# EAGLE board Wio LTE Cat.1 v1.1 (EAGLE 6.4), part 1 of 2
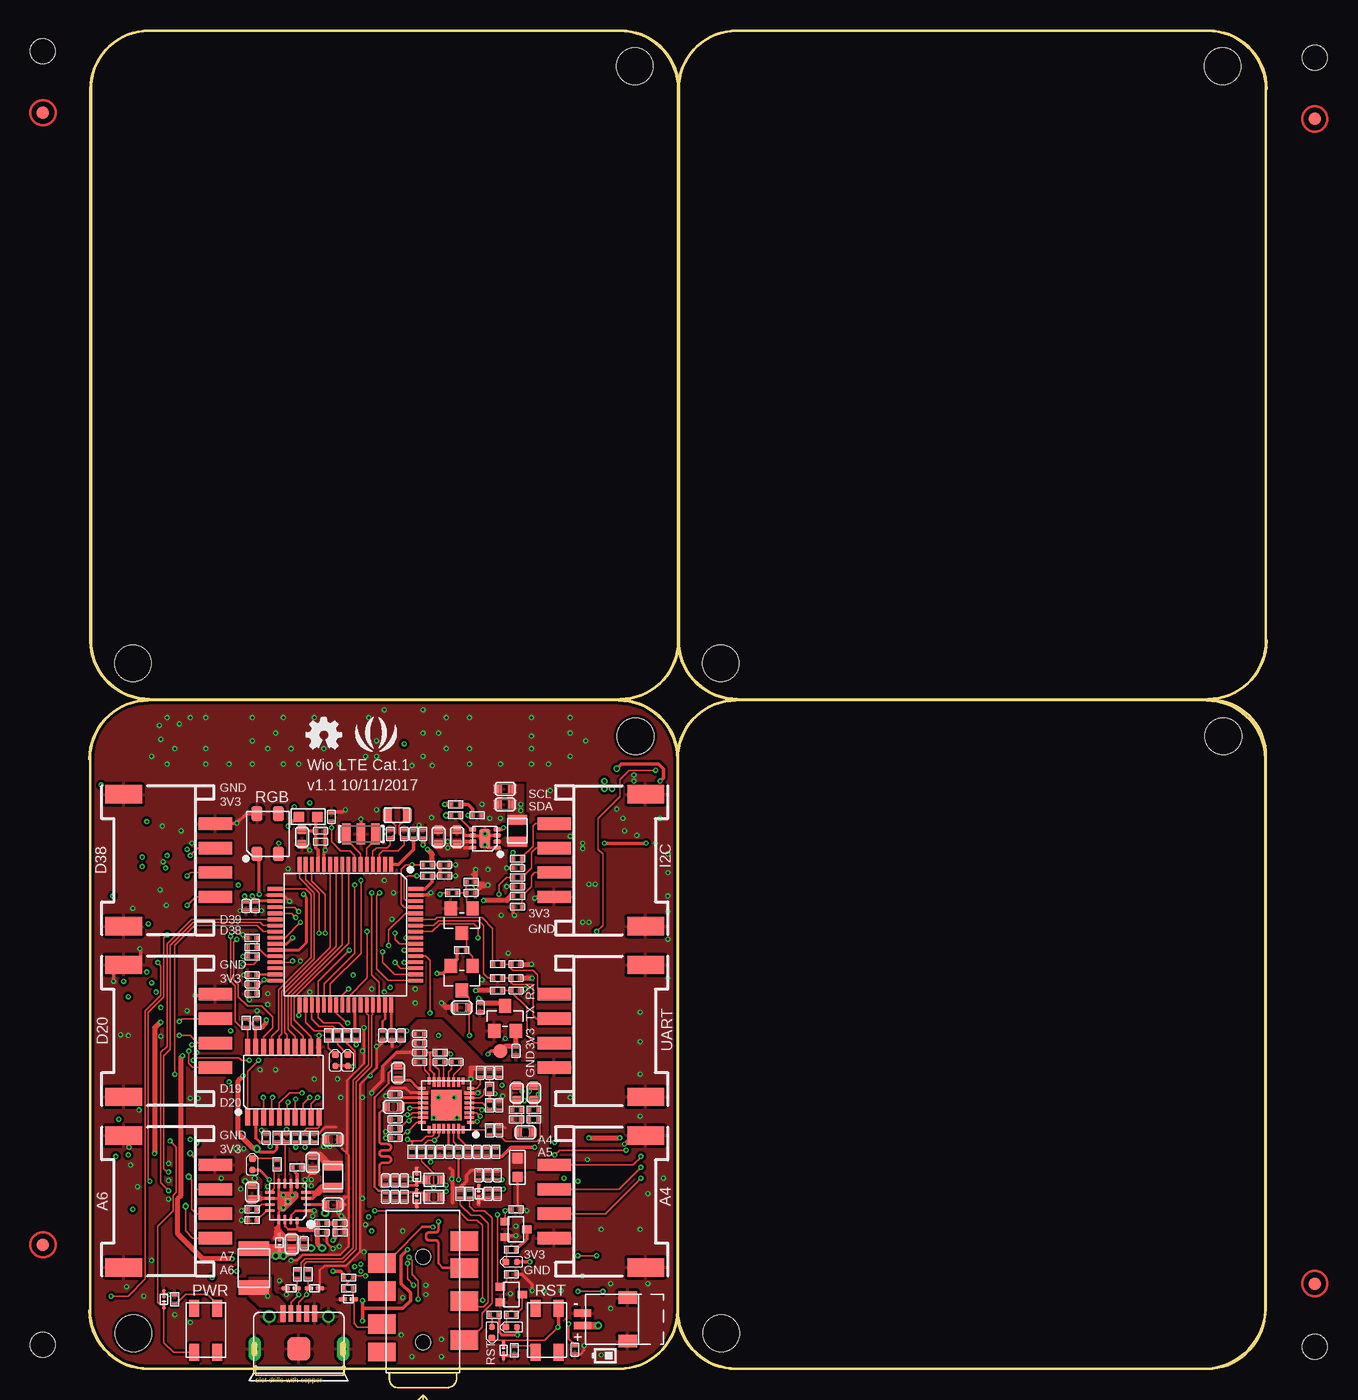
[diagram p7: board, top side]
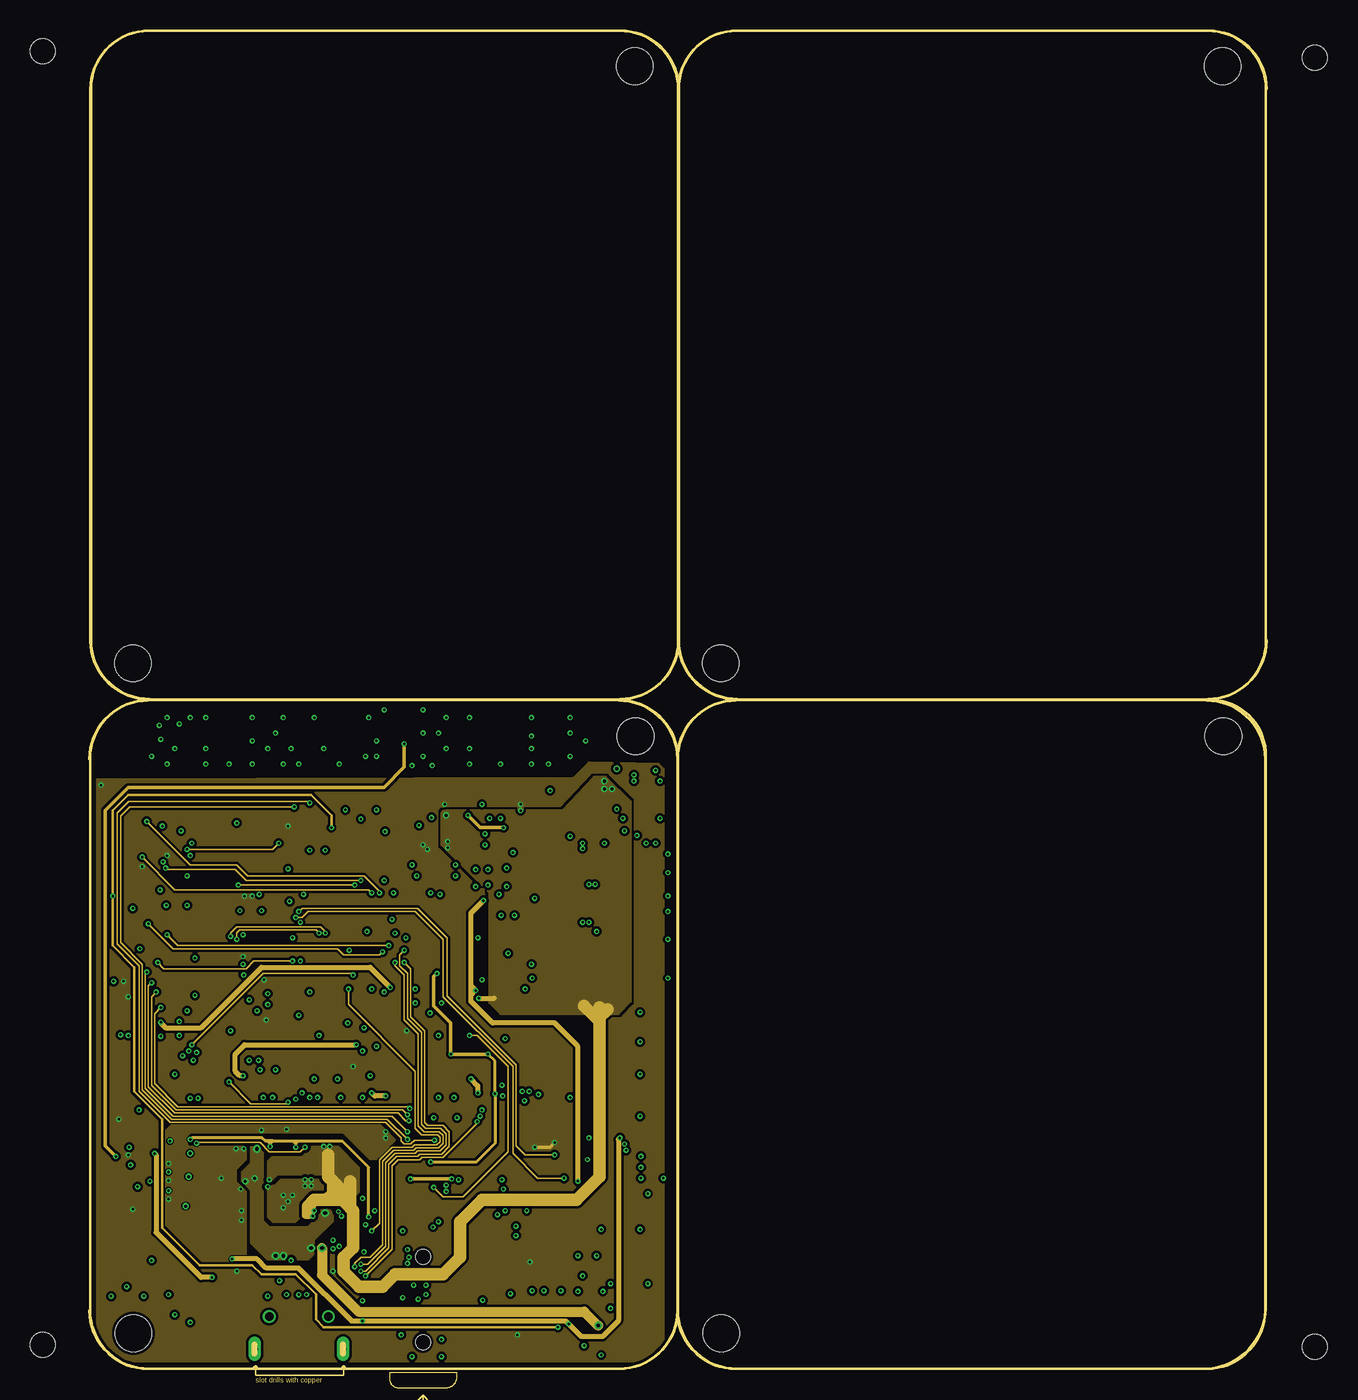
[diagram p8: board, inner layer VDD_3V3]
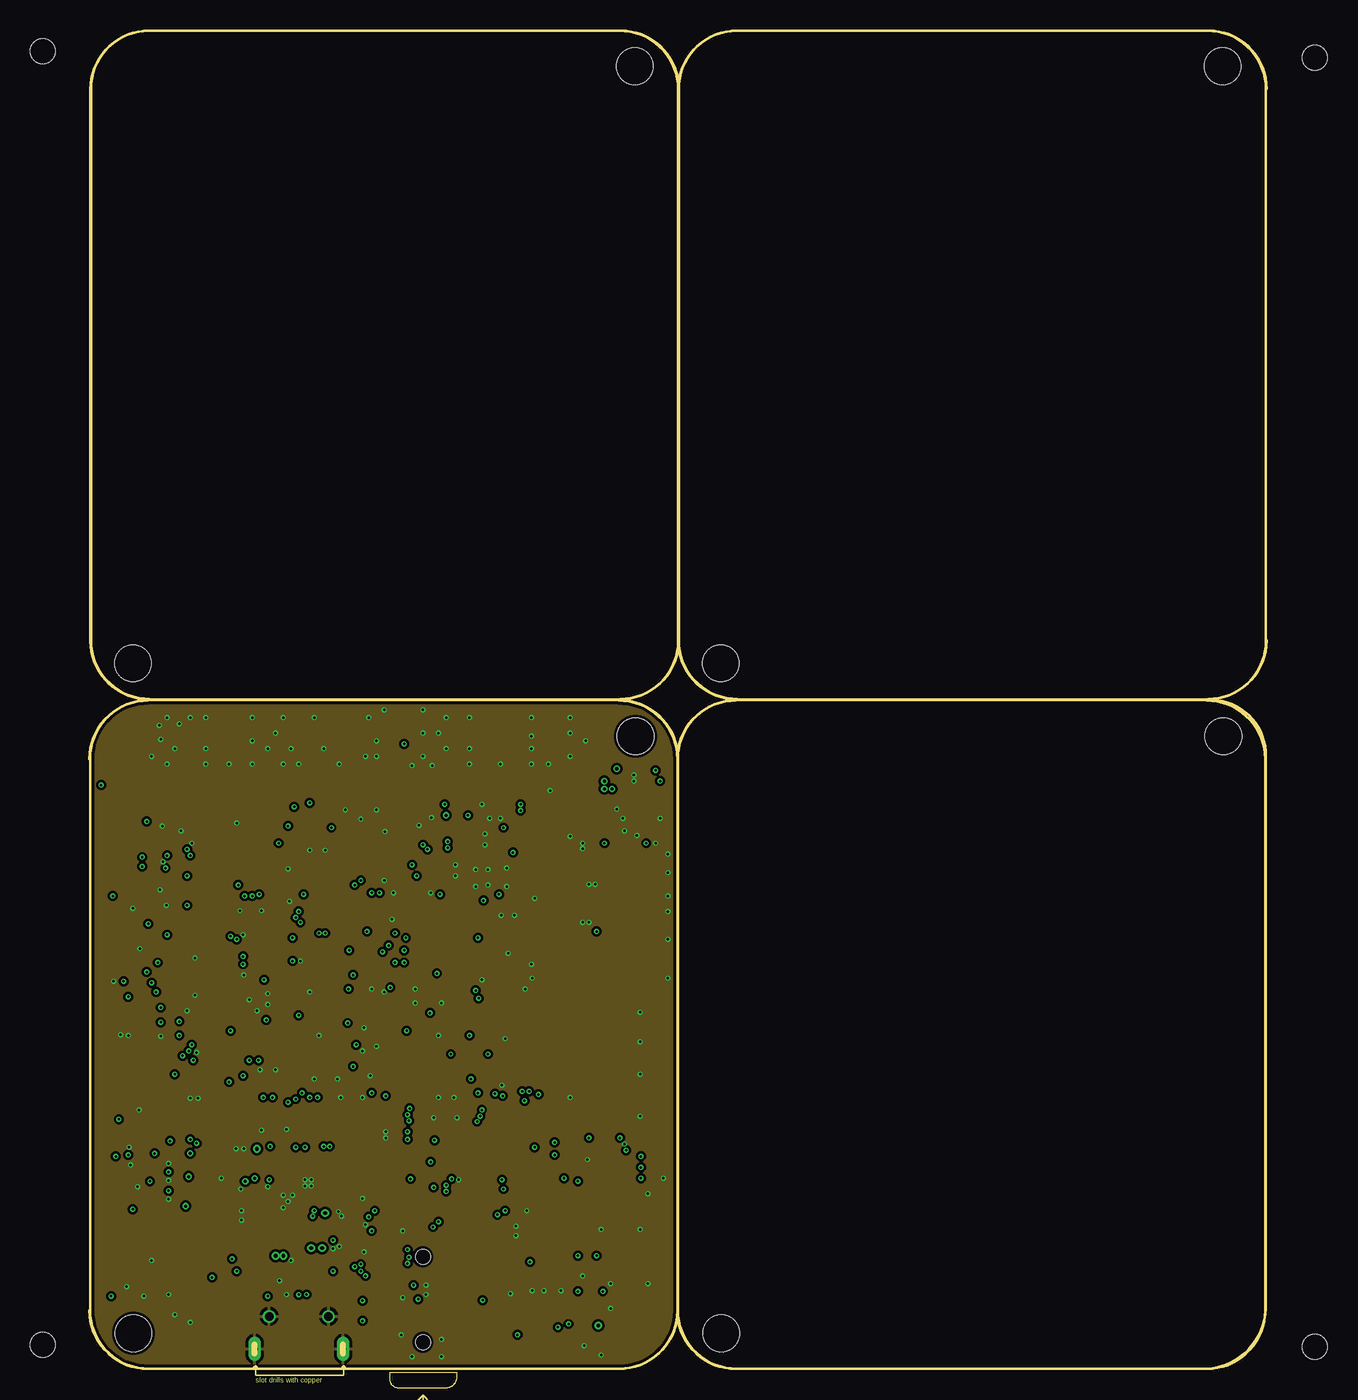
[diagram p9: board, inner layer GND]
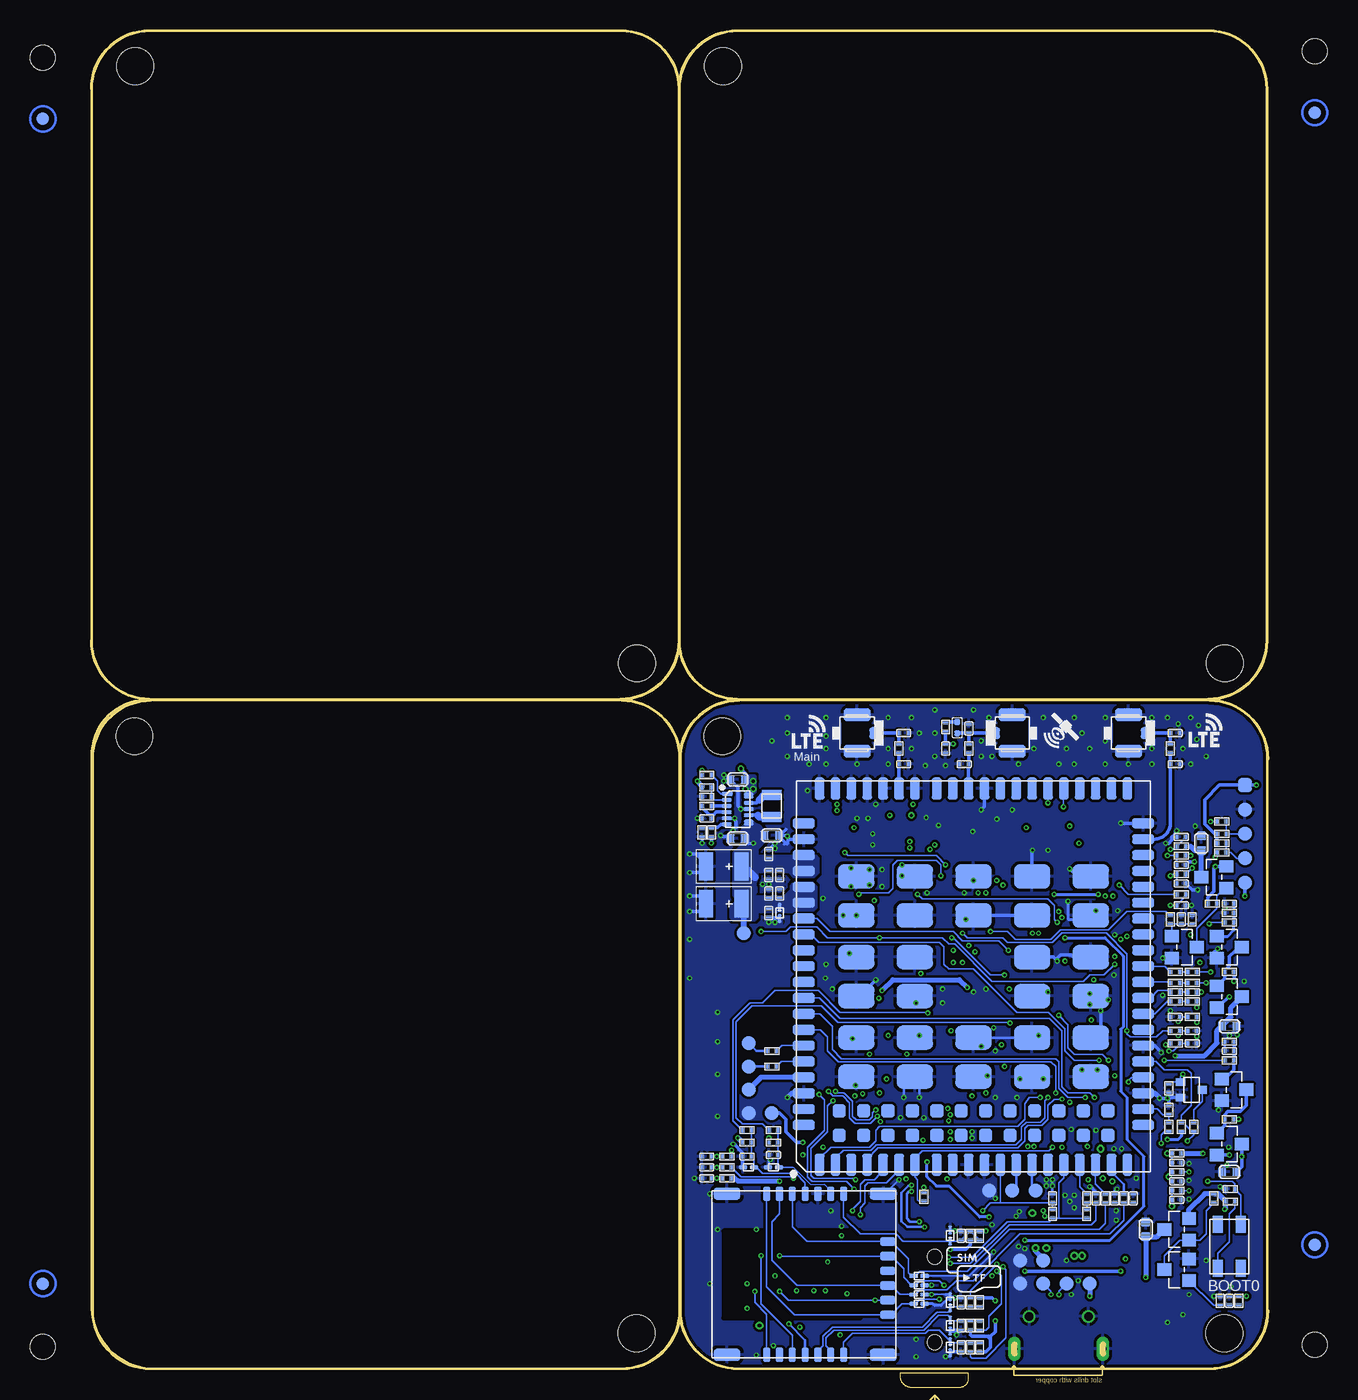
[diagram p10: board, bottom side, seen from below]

Size 96.39 x 109.6 mm. Coordinates in mm from the lower left corner, seen from the top.
Outline: 71 segments
Copper layers (1*2*15*16): Top 0.035mm / dielectric 0.2mm / VDD_3V3 0.0175mm / dielectric 0.3mm / GND 0.0175mm / dielectric 0.2mm / Bottom 0.035mm
Design rules "SeeedStudio_4layer_DRU_no_angle_20140221 *": minimum track width 1mil, minimum drill 8mil, track to track 4mil, track to pad 4mil, pad to pad 4mil, via to via 4mil, smd to smd 0mil, copper to edge 10mil, drill to drill 8mil, minimum pad ring 3mil, minimum via ring 3mil, stop-mask expansion 4mil, vias tented up to drill 25mil, thermal gap 10mil
Holes 3 mm at 3.6,2.92 44.7,51.82 51.74,2.92 92.84,51.82 92.79,106.68 51.69,57.78 44.66,106.68 3.56,57.78
Holes 2.03 mm at -3.81,1.98 -3.81,107.9 100.33,107.36 100.33,1.83
tRestrict: area 31.1,31.4 to 31.9,32.8; area 19.2,15.4 to 20.7,16.1; area 34.3,43.8 to 35.8,44.3
bRestrict: area 39.9,45.7 to 41.3,46.5; area 32.1,47.4 to 32.4,47.8; area 33.3,47.4 to 33.7,47.8; area 34.5,47.4 to 35.1,47.6; area 35.9,47.4 to 36.2,47.6; area 23.7,16.5 to 24,16.9

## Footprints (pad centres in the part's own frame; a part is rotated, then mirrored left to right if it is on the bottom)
U-FL3P-SMD-2.6X2.6X1.0MM = smd 1.05 x 1: D -1.524,0 | smd 2.2 x 1.05: GND1 0,1.5; GND2 0,-1.5
C0402 = smd 0.508 x 0.385: 1 0,0.383; 2 0,-0.383
C0603 = smd 0.762 x 0.696: 1 0,0.602; 2 0,-0.602
AVX-B = smd 1.143 x 2.286: + -1.46,0; - 1.46,0
SOD-923 = smd 0.7 x 0.3: 1 -0.45,0; 2 0.45,0
LED-0402 = smd 0.5 x 0.5: + -0.463,0 | smd 0.58 x 0.58: - 0.468,0
F1210 = smd 1.2 x 2.5: 1 -1.6,0; 2 1.6,0
HW2-SMD-1.0-90D = smd 1.524 x 1.016: 3 -3.429,1.778; 4 -3.429,-1.778 | smd 1.397 x 0.635: + 0.254,0.508; - 0.254,-0.508
SIM+TF-24P-SMD-1.2-15.05X13.66X2.5MM = smd 1.2 x 0.6: P1 0,3.26; P2 0,4.31; P3 0,5.36; P5 13.2,3.26; P6 13.2,4.31; P7 13.2,5.36; T1 13.2,9.56; T2 13.2,8.51; T3 13.2,7.46; T4 13.2,6.41; T5 0,6.41; T6 0,7.46; T7 0,8.51; T8 0,9.56 | smd 0.7 x 1.2: P1B 9.91,13.17; P2B 7.51,13.17; P3B 3.91,13.17; P5B 8.71,13.17; P6B 6.31,13.17; P7B 5.11,13.17 | smd 1 x 2.2: PAD 0,0; PAD1 0,12.8; PAD2 13.2,0; PAD3 13.2,12.8
AUDIO8P-SMD-3.5-14.5X6.1X4.0MM = smd 1.6 x 2.25: 1 3.9,-3.375; 2 7.1,-3.375; 3 9.8,-3.375; 4 10.2,3.375; 6 5.2,3.375; 7 7.9,3.375; 8 12,-3.375 | smd 1.5 x 2.25: 5 2.9,3.375 | hole 1.2: 3.7,0; 10.7,0
H5-SMD-2.0-TEST = smd 1.143 x 1.143: 1 0,4; 2 0,2; 3 0,0; 4 0,-2; 5 0,-4
MICRO-USB5+5P-SMD-0.65-7.2X5.06MM = smd 0.4 x 1.35: 1 -1.3,2.875; 2 -0.65,2.875; 3 0,2.875; 4 0.65,2.875; 5 1.3,2.875 | smd 1.9 x 1.9: P1 0,0 | drill 0.508 pad 1.016 long: P3 -3.625,0; P4 3.625,0 | drill 0.7: P5 -2.425,2.65; P6 2.425,2.65
HW4-SMD-2.0-90D = smd 1.01 x 2.74: 1 -3,-0.1; 2 -1,-0.1; 3 1,-0.1; 4 3,-0.1 | smd 1.5 x 3: SS1 -5.4,7.4; SS2 5.4,7.4
SW4P-SMD-4.5X3.2X2.5MM = smd 1.4 x 0.8: 1 -1.8,-0.94; 2 1.8,-0.94; 3 1.8,0.94; 4 -1.8,0.94
L0402 = smd 0.5 x 0.5: 1 -0.463,0; 2 0.463,0
L201610 = smd 0.8 x 1.6: 1 -0.9,0; 2 0.9,0
L0603 = smd 0.889 x 0.889: 1 -0.762,0; 2 0.762,0
LED4-1.75-3.7X3.5X0.95MM = smd 1.2 x 0.9: 1 -1.65,0.875; 2 -1.65,-0.875; 3 1.65,-0.875; 4 1.65,0.875
ROUND-MARK-1.0 = smd 1.016 x 1.016: P$1 0,0
SOT-323 = smd 0.635 x 0.762: 1 -0.635,-0.889; 2 0.635,-0.889; 3 0,0.889
SOT-23 = smd 1.016 x 1.143: 1 -0.889,-1.016; 2 0.889,-1.016; 3 0,1.016
R0402 = smd 0.508 x 0.385: 1 0,0.383; 2 0,-0.383
R0603 = smd 0.762 x 0.696: 1 0,0.602; 2 0,-0.602
R0603' = smd 0.889 x 0.889: 1 0,0.762; 2 0,-0.762
TP-D45MIL = smd 1.143 x 1.143: T 0,0
MODULE144P-1.3-32X29X2.4MM = smd 1.8 x 0.8: 1 -15.4,12.6; 2 -15.4,11.3; 3 -15.4,10; 4 -15.4,8.7; 5 -15.4,7.4; 6 -15.4,6.1; 7 -15.4,4.8; 8 -15.4,0.4; 9 -15.4,-0.9; 10 -15.4,-2.2; 11 -15.4,-3.5; 12 -15.4,-4.8; 13 -15.4,-6.1; 14 -15.4,-7.4; 15 -15.4,-8.7; 16 -15.4,-10; 17 -15.4,-11.3; 18 -15.4,-12.6; 37 15.4,-12.6; 38 15.4,-11.3; 39 15.4,-10; 40 15.4,-8.7; 41 15.4,-7.4; 42 15.4,-6.1; 43 15.4,-4.8; 44 15.4,-3.5; 45 15.4,-2.2; 46 15.4,-0.9; 47 15.4,0.4; 48 15.4,4.8; 49 15.4,6.1; 50 15.4,7.4; 51 15.4,8.7; 52 15.4,10; 53 15.4,11.3; 54 15.4,12.6; 141 -15.4,3; 142 -15.4,1.7; 143 15.4,1.7; 144 15.4,3 | smd 0.8 x 1.8: 19 -9.55,-13.9; 20 -8.25,-13.9; 21 -6.95,-13.9; 22 -5.65,-13.9; 23 -4.35,-13.9; 24 -3.05,-13.9; 25 -1.75,-13.9; 26 -0.45,-13.9; 27 0.85,-13.9; 28 2.15,-13.9; 29 3.45,-13.9; 30 4.75,-13.9; 31 6.05,-13.9; 32 7.35,-13.9; 33 8.65,-13.9; 34 9.95,-13.9; 35 11.25,-13.9; 36 12.55,-13.9; 55 12.55,13.9; 56 11.25,13.9; 57 9.95,13.9; 58 8.65,13.9; 59 7.35,13.9; 60 6.05,13.9; 61 4.75,13.9; 62 3.45,13.9; 63 2.15,13.9; 64 0.85,13.9; 65 -0.45,13.9; 66 -1.75,13.9; 67 -3.05,13.9; 68 -4.35,13.9; 69 -5.65,13.9; 70 -6.95,13.9; 71 -8.25,13.9; 72 -9.55,13.9; 113 -10.85,13.9; 114 -12.15,13.9; 115 -10.85,-13.9; 116 -12.15,-13.9 | smd 2 x 3: 85 8.2,9.6; 86 8.2,4.8; 87 8.2,0; 88 8.2,-4.8; 89 8.2,-9.6; 90 5,9.6; 91 5,4.8; 92 5,0; 93 5,-4.8; 94 5,-9.6; 95 1.6,9.6; 96 1.6,4.8; 97 1.6,-4.8; 98 1.6,-9.6; 99 -1.6,9.6; 100 -1.6,4.8; 101 -1.6,-4.8; 102 -1.6,-9.6; 103 -5,9.6; 104 -5,4.8; 105 -5,0; 106 -5,-4.8; 107 -5,-9.6; 108 -8.2,9.6; 109 -8.2,4.8; 110 -8.2,0; 111 -8.2,-4.8; 112 -8.2,-9.6 | smd 1.1 x 1.1: 117 -11,11; 118 -11,9; 119 -11,7; 120 -11,5; 121 -11,3; 122 -11,1; 123 -11,-1; 124 -11,-3; 125 -11,-5; 126 -11,-7; 127 -11,-9; 128 -11,-11; 129 -13,11; 130 -13,9; 131 -13,7; 132 -13,5; 133 -13,3; 134 -13,1; 135 -13,-1; 136 -13,-3; 137 -13,-5; 138 -13,-7; 139 -13,-9; 140 -13,-11
LQFP64 = smd 0.3 x 1.2: 1 -3.75,-5.75; 2 -3.25,-5.75; 3 -2.75,-5.75; 4 -2.25,-5.75; 5 -1.75,-5.75; 6 -1.25,-5.75; 7 -0.75,-5.75; 8 -0.25,-5.75; 9 0.25,-5.75; 10 0.75,-5.75; 11 1.25,-5.75; 12 1.75,-5.75; 13 2.25,-5.75; 14 2.75,-5.75; 15 3.25,-5.75; 16 3.75,-5.75; 33 3.75,5.75; 34 3.25,5.75; 35 2.75,5.75; 36 2.25,5.75; 37 1.75,5.75; 38 1.25,5.75; 39 0.75,5.75; 40 0.25,5.75; 41 -0.25,5.75; 42 -0.75,5.75; 43 -1.25,5.75; 44 -1.75,5.75; 45 -2.25,5.75; 46 -2.75,5.75; 47 -3.25,5.75; 48 -3.75,5.75 | smd 1.2 x 0.3: 17 5.75,-3.75; 18 5.75,-3.25; 19 5.75,-2.75; 20 5.75,-2.25; 21 5.75,-1.75; 22 5.75,-1.25; 23 5.75,-0.75; 24 5.75,-0.25; 25 5.75,0.25; 26 5.75,0.75; 27 5.75,1.25; 28 5.75,1.75; 29 5.75,2.25; 30 5.75,2.75; 31 5.75,3.25; 32 5.75,3.75; 49 -5.75,3.75; 50 -5.75,3.25; 51 -5.75,2.75; 52 -5.75,2.25; 53 -5.75,1.75; 54 -5.75,1.25; 55 -5.75,0.75; 56 -5.75,0.25; 57 -5.75,-0.25; 58 -5.75,-0.75; 59 -5.75,-1.25; 60 -5.75,-1.75; 61 -5.75,-2.25; 62 -5.75,-2.75; 63 -5.75,-3.25; 64 -5.75,-3.75
QFN32G-0.4-4X4MM = smd 0.6 x 0.25: 1 -2,1.4; 8 -2,-1.4; 17 2,-1.4; 24 2,1.4 | smd 0.8 x 0.25: 2 -1.9,1; 3 -1.9,0.6; 4 -1.9,0.2; 5 -1.9,-0.2; 6 -1.9,-0.6; 7 -1.9,-1; 18 1.9,-1; 19 1.9,-0.6; 20 1.9,-0.2; 21 1.9,0.2; 22 1.9,0.6; 23 1.9,1 | smd 0.25 x 0.6: 9 -1.4,-2; 16 1.4,-2; 25 1.4,2; 32 -1.4,2 | smd 0.25 x 0.8: 10 -1,-1.9; 11 -0.6,-1.9; 12 -0.2,-1.9; 13 0.2,-1.9; 14 0.6,-1.9; 15 1,-1.9; 26 1,1.9; 27 0.6,1.9; 28 0.2,1.9; 29 -0.2,1.9; 30 -0.6,1.9; 31 -1,1.9 | smd 2.5 x 2.5: PAD 0,0
QFN16G-0.5-3X3MM@1 = smd 0.65 x 0.28: 1 -1.575,0.75; 2 -1.575,0.25 | smd 0.85 x 0.28: 3 -1.475,-0.25; 4 -1.475,-0.75; 9 1.475,-0.75; 10 1.475,-0.25; 11 1.475,0.25; 12 1.475,0.75 | smd 0.28 x 0.85: 5 -0.75,-1.475; 6 -0.25,-1.475; 7 0.25,-1.475; 8 0.75,-1.475; 13 0.75,1.475; 14 0.25,1.475 | smd 0.28 x 0.65: 15 -0.25,1.575; 16 -0.75,1.575 | smd 0.508 x 0.508: PAD 0,0
DFN8G-0.5-2X2MM = smd 0.6 x 0.3: 1 -1,0.75; 2 -1,0.25; 3 -1,-0.25; 4 -1,-0.75; 5 1,-0.75; 6 1,-0.25; 7 1,0.25; 8 1,0.75 | smd 0.9 x 1.6: 9 0,0
QFN11-0.5-2X3MM = smd 0.9 x 0.3: 1 -0.85,1.25 | smd 0.8 x 0.3: 2 -0.9,0.75; 3 -0.9,0.25; 4 -0.9,-0.25; 5 -0.9,-0.75; 6 -0.9,-1.25; 8 0.9,-0.5; 9 0.9,0; 10 0.9,0.5 | smd 0.8 x 0.5: 7 0.9,-1.1; 11 0.9,1.1
TSSOP20-0.65-6.5X4.4MM = smd 0.4 x 1.35: 1 -2.925,-2.875; 2 -2.275,-2.875; 3 -1.625,-2.875; 4 -0.975,-2.875; 5 -0.325,-2.875; 6 0.325,-2.875; 7 0.975,-2.875; 8 1.625,-2.875; 9 2.275,-2.875; 10 2.925,-2.875; 11 2.91,2.875; 12 2.26,2.875; 13 1.61,2.875; 14 0.96,2.875; 15 0.325,2.875; 16 -0.325,2.875; 17 -0.975,2.875; 18 -1.625,2.875; 19 -2.275,2.875; 20 -2.925,2.875
X2-SMD-L2.0X1.2X0.55MM = smd 0.762 x 1.143: 1 -0.813,0; 2 0.813,0
RESONATOR3-SMD-3.6X1.3X0.8MM = smd 0.7 x 1.7: 1 -1.2,0; 2 0,0; 3 1.2,0

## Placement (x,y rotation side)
ANT1  [U-FL3P-SMD-2.6X2.6X1.0MM]  11.43,52.07 180 bottom
ANT2  [U-FL3P-SMD-2.6X2.6X1.0MM]  20.95,52.07 0 bottom
ANT4  [U-FL3P-SMD-2.6X2.6X1.0MM]  33.66,52.07 180 bottom
C1  4.7uF  [C0402]  13.34,32.26 90 top
C2  10uF  [C0402]  32,29.59 180 top
C3  10uF  [C0603]  19.94,13.46 90 top
C4  10uF  [C0603]  13.34,14.48 0 top
C5  100nF  [C0402]  40.01,38.93 0 bottom
C6  33pF  [C0402]  25.15,10.92 180 bottom
C7  100nF  [C0402]  17.59,10.29 0 top
C8  10uF  [C0603]  16.57,10.22 0 top
C9  DNP  [C0402]  29.84,49.53 270 bottom
C10  22pF  [C0402]  25.78,43.81 180 top
C11  22pF  [C0402]  24.64,43.81 180 top
C12  33pF  [C0402]  25.15,1.78 0 bottom
C13  22uF  [C0603]  43.43,48.26 90 bottom
C14  10pF  [C0402]  40.89,37.34 180 bottom
C15  22uF  [C0603]  40.64,43.69 90 bottom
C16  100nF  [C0402]  39.75,1.59 180 top
C17  33pF  [C0402]  25.15,5.46 180 bottom
C18  33pF  [C0402]  42.67,17.4 270 bottom
C19  33pF  [C0402]  14.1,13.97 180 bottom
C20  33pF  [C0402]  12.57,13.97 180 bottom
C21  33pF  [C0402]  11.05,13.97 180 bottom
C22  1uF  [C0402]  7.11,43.56 90 bottom
C23  100nF  [C0402]  19.81,45.21 180 top
C24  22uF  [C0603]  18.29,16.89 0 top
C25  1uF  [C0402]  19.05,11.18 90 top
C26  2.2uF  [C0402]  30.04,25.15 90 top
C27  2.2uF  [C0402]  28.7,25.15 90 top
C28  1uF  [C0603]  24.89,21.46 270 top
C29  1uF  [C0603]  25.27,24.26 180 top
C30  100nF  [C0402]  13.59,37.91 180 top
C31  1uF  [C0402]  12.83,37.91 180 top
C32  100nF  [C0402]  13.34,31.5 90 top
C33  2.2uF  [C0402]  25.02,22.48 270 top
C34  DNP  [C0402]  29.84,52.07 270 bottom
C35  4.7uF  [C0402]  27.05,27.43 90 top
C36  2.2uF  [C0402]  27.05,25.15 270 top
C37  4.7uF  [C0402]  33.53,19.56 0 top
C38  1uF  [C0402]  27.3,43.81 0 top
C39  100nF  [C0402]  26.54,43.81 0 top
C40  DNP  [C0402]  25.02,18.92 270 top
C41  DNP  [C0402]  25.02,19.68 270 top
C42  4.7uF  [C0402]  32,24.26 0 top
C43  100nF  [C0402]  27.05,26.67 90 top
C44  DNP  [C0402]  25.02,20.45 270 top
C45  33pF  [C0402]  27.05,25.91 90 top
C46  2.2uF  [C0402]  30.23,17.78 0 top
C47  2.2uF  [C0402]  28.7,17.78 180 top
C48  100nF  [C0402]  29.46,17.78 0 top
C49  4.7uF  [C0402]  32.51,17.78 180 top
C50  100nF  [C0402]  31.75,17.78 180 top
C51  33pF  [C0402]  30.99,17.78 180 top
C52  4.7uF  [C0402]  33.53,24.26 0 top
C53  100nF  [C0402]  32.77,24.26 0 top
C54  4.7uF  [C0402]  33.53,21.59 0 top
C55  22uF  [C0603]  43.43,43.43 270 bottom
C56  1uF  [C0402]  45.97,45.09 90 bottom
C57  33pF  [C0402]  7.11,39.75 90 bottom
C58  100nF  [C0402]  17.65,12.7 180 bottom
C59  33pF  [C0402]  17.65,13.97 180 bottom
C60  33pF  [C0402]  40.51,17.53 270 bottom
C61  33pF  [C0402]  25.15,3.56 0 bottom
C62  33pF  [C0402]  7.11,37.97 90 bottom
C63  33pF  [C0402]  7.11,41.27 90 bottom
C64  33pF  [C0402]  6.22,27.69 90 bottom
C65  100nF  [C0402]  14.48,18.92 0 top
C66  100nF  [C0402]  29.08,40.39 270 top
C67  100nF  [C0402]  7.11,36.83 180 bottom
C68  1uF  [C0402]  13.34,30.73 90 top
C70  100nF  [C0402]  24.77,27.3 180 top
C71  1uF  [C0402]  25.53,27.3 180 top
C74  33pF  [C0402]  40.89,38.93 0 bottom
C75  100nF  [C0402]  29.08,41.27 270 top
C76  1uF  [C0402]  13.72,28.32 0 top
C77  220uF  [AVX-B]  44.58,38.1 180 bottom
C78  100nF  [C0402]  20.51,11.94 90 top
C79  10uF  [C0603]  3.17,28.07 90 bottom
C80  10uF  [C0603]  35.69,19.37 90 top
C81  2.2uF  [C0603]  36.39,22.61 180 top
C82  2.2uF  [C0603]  34.99,22.61 180 top
C83  4.7uF  [C0402]  33.4,15.88 0 top
C84  10pF  [C0402]  31.88,15.88 0 top
C85  33pF  [C0402]  32.64,15.88 0 top
C86  33pF  [C0402]  24.26,14.1 180 top
C87  10pF  [C0402]  25.02,15.43 180 top
C88  33pF  [C0402]  24.26,15.43 0 top
C89  10pF  [C0402]  25.02,14.1 180 top
C90  33pF  [C0402]  33.4,14.35 180 top
C91  100nF  [C0402]  3.17,38.1 270 bottom
C92  10uF  [C0603]  3.17,16.13 270 bottom
C93  100nF  [C0402]  3.17,26.04 270 bottom
C94  10pF  [C0402]  32.64,14.35 180 top
C95  DNP  [C0402]  7.62,49.53 270 bottom
C96  DNP  [C0402]  25.78,15.43 180 top
C97  DNP  [C0402]  25.78,14.1 180 top
C98  DNP  [C0402]  7.62,52.07 270 bottom
C99  DNP  [C0402]  24.89,49.53 90 bottom
C100  DNP  [C0402]  24.51,52.45 0 bottom
C101  DNP  [C0402]  26.42,50.8 180 bottom
C102  10uF  [C0603]  34.04,46.23 90 top
C103  10uF  [C0603]  28.57,43.56 0 top
C104  10uF  [C0603]  34.04,47.5 90 top
C105  10uF  [C0603]  30.1,43.56 0 top
C106  100nF  [C0402]  40.89,42.16 0 bottom
C107  10pF  [C0402]  40.89,40.45 180 bottom
C112  33pF  [C0402]  40.01,40.45 180 bottom
C113  220uF  [AVX-B]  44.58,41.15 180 bottom
C114  33pF  [C0402]  7.62,28.83 270 bottom
C115  33pF  [C0402]  6.22,26.67 90 bottom
C116  33pF  [C0402]  7.49,15.37 90 bottom
C117  33pF  [C0402]  7.49,16.89 90 bottom
C118  1uF  [C0402]  18.92,43.18 270 top
C119  100nF  [C0402]  18.92,44.07 270 top
C120  10uF  [C0402]  34.92,26.04 180 top
C125  4.7uF  [C0402]  24,27.3 180 top
C126  33pF  [C0402]  7.49,13.84 90 bottom
C127  33pF  [C0402]  34.92,32 90 top
C128  33pF  [C0402]  34.92,30.99 90 top
C129  33pF  [C0402]  34.92,33.15 90 top
C130  33pF  [C0402]  45.97,16.51 270 bottom
C131  33pF  [C0402]  45.97,15.62 270 bottom
C132  33pF  [C0402]  45.97,17.4 270 bottom
C133  33pF  [C0402]  35.05,39.5 270 top
C134  33pF  [C0402]  35.05,37.85 270 top
C135  33pF  [C0402]  35.05,41.02 270 top
C136  10uF  [C0603]  10.03,11.43 180 bottom
C137  100nF  [C0402]  3.17,5.59 180 bottom
C138  22uF  [C0603]  19.94,18.8 90 top
C139  22uF  [C0603]  17.4,43.56 0 top
C140  10uF  [C0603]  5.46,43.05 180 bottom
C142  10uF  [C0603]  30.48,29.59 270 top
C143  100nF  [C0402]  31.24,38.99 90 top
D1  DF2S6.8FS  [SOD-923]  15.56,10.35 90 top
D3  DF2S6.8FS  [SOD-923]  16.51,6.6 180 top
D5  DF2S6.8FS  [SOD-923]  18.41,6.6 0 top
D6  GREEN  [LED-0402]  21.15,25.27 90 top
D7  ESD;DF2S6.8FS  [SOD-923]  26.04,1.78 270 bottom
D8  ESD;DF2S6.8FS  [SOD-923]  28.57,6.86 0 bottom
D9  ESD;DF2S6.8FS  [SOD-923]  26.8,15.75 90 top
D10  ESD;DF2S6.8FS  [SOD-923]  28.57,7.62 0 bottom
D11  ESD;DF2S6.8FS  [SOD-923]  28.57,6.1 0 bottom
D12  ESD;DF2S6.8FS  [SOD-923]  28.57,5.33 0 bottom
D13  ESD;DF2S6.8FS  [SOD-923]  26.8,13.97 270 top
D14  RED  [LED-0402]  32.96,2.98 270 top
D15  ESD;DF2S6.8FS  [SOD-923]  31.88,14.35 270 top
D16  GREEN  [LED-0402]  13.34,16.76 90 top
D17  GREEN  [LED-0402]  20.13,25.27 90 top
D18  ESD;DF2S6.8FS  [SOD-923]  21.21,5.71 180 top
D19  ESD;DF2S6.8FS  [SOD-923]  40.51,16.51 180 bottom
D20  ESD;DF2S6.8FS  [SOD-923]  42.55,16.51 180 bottom
D21  ESD;DF2S6.8FS  [SOD-923]  26.04,10.92 90 bottom
D22  ESD;DF2S6.8FS  [SOD-923]  26.04,5.46 90 bottom
D23  ESD;DF2S6.8FS  [SOD-923]  26.04,3.56 270 bottom
D24  RED  [LED-0402]  34.54,3.43 180 top
D25  RED  [LED-0402]  34.54,8.76 180 top
D26  ESD;DF2S6.8FS  [SOD-923]  6.1,5.71 90 top
D27  ESD;DF2S6.8FS  [SOD-923]  33.91,1.52 270 top
D28  DNP  [SOD-923]  40.01,37.34 270 bottom
F1  2A/6V  [F1210]  13.46,8.26 90 top
FR1  SEEEDSTUDIO-OPEN-SCH-FRAME  [SEEEDSTUDIO-PCB-FRAME]  not placed on the board
FR2  SEEEDSTUDIO-OPEN-SCH-FRAME  [SEEEDSTUDIO-PCB-FRAME]  not placed on the board
FR3  SEEEDSTUDIO-OPEN-SCH-FRAME  [SEEEDSTUDIO-PCB-FRAME]  not placed on the board
FR4  SEEEDSTUDIO-OPEN-SCH-FRAME  [SEEEDSTUDIO-PCB-FRAME]  not placed on the board
FR5  SEEEDSTUDIO-OPEN-SCH-FRAME  [SEEEDSTUDIO-PCB-FRAME]  not placed on the board
FR6  SEEEDSTUDIO-OPEN-SCH-FRAME  [SEEEDSTUDIO-PCB-FRAME]  not placed on the board
FR7  SEEEDSTUDIO-OPEN-SCH-FRAME  [SEEEDSTUDIO-PCB-FRAME]  not placed on the board
FR8  SEEEDSTUDIO-OPEN-SCH-FRAME  [SEEEDSTUDIO-PCB-FRAME]  not placed on the board
FR9  SEEEDSTUDIO-OPEN-SCH-FRAME  [SEEEDSTUDIO-PCB-FRAME]  not placed on the board
FR10  SEEEDSTUDIO-OPEN-SCH-FRAME  [SEEEDSTUDIO-PCB-FRAME]  not placed on the board
J1  JST-2P-SMD-90D  [HW2-SMD-1.0-90D]  40.64,4.06 180 top
J2  [SIM+TF-24P-SMD-1.2-15.05X13.66X2.5MM]  44.32,14.35 270 bottom
J3  [AUDIO8P-SMD-3.5-14.5X6.1X4.0MM]  27.3,-1.52 90 top
J4  [H5-SMD-2.0-TEST]  1.91,43.81 0 bottom
J10  USB  [MICRO-USB5+5P-SMD-0.65-7.2X5.06MM]  17.14,1.65 0 top
J11  D38  [HW4-SMD-2.0-90D]  10.21,41.66 90 top
J12  D20  [HW4-SMD-2.0-90D]  10.21,27.69 90 top
J13  A6  [HW4-SMD-2.0-90D]  10.21,13.72 90 top
J14  I2C  [HW4-SMD-2.0-90D]  38.15,41.66 270 top
J15  URAT  [HW4-SMD-2.0-90D]  38.15,27.69 270 top
J16  A4  [HW4-SMD-2.0-90D]  38.15,13.72 270 top
K1  KEY  [SW4P-SMD-4.5X3.2X2.5MM]  3.17,10.03 270 bottom
K3  KEY  [SW4P-SMD-4.5X3.2X2.5MM]  37.47,3.17 90 top
K4  KEY  [SW4P-SMD-4.5X3.2X2.5MM]  9.53,3.17 270 top
L1  47nH  [L0402]  25.46,52.51 90 bottom
L2  470nH  [L201610]  35.05,44.07 90 top
L3  1uH  [L201610]  40.64,46.1 270 bottom
L6  2.2uH  [L201610]  19.94,15.75 90 top
L12  30R/3000mA  [L0603]  17.91,45.21 0 top
LED2  RGB-SK6812MINI  [LED4-1.75-3.7X3.5X0.95MM]  14.61,43.81 270 top
P1  [ROUND-MARK-1.0]  not placed on the board
P2  [ROUND-MARK-1.0]  not placed on the board
P3  [ROUND-MARK-1.0]  not placed on the board
P4  [ROUND-MARK-1.0]  not placed on the board
P5  [ROUND-MARK-1.0]  not placed on the board
P6  [ROUND-MARK-1.0]  not placed on the board
P7  [ROUND-MARK-1.0]  not placed on the board
P8  [ROUND-MARK-1.0]  not placed on the board
Q1  2N7002KW  [SOT-323]  6.29,22.86 270 bottom
Q2  CJ3407A  [SOT-23]  7.49,11.43 90 bottom
Q3  2N7002  [SOT-23]  7.49,8.13 90 bottom
Q4  CJ3407A  [SOT-23]  4.45,40.26 90 bottom
Q5  2N7002  [SOT-23]  6.86,34.54 270 bottom
Q6  CJ3407A  [SOT-23]  30.48,32 180 top
Q7  2N7002  [SOT-23]  30.48,36.7 180 top
Q9  2N7002KW  [SOT-323]  34.54,6.1 270 top
Q10  2N7002KW  [SOT-323]  34.92,11.43 270 top
Q13  CJ3407A  [SOT-23]  3.17,30.48 270 bottom
Q14  2N7002  [SOT-23]  3.17,34.54 270 bottom
Q15  CJ3407A  [SOT-23]  3.17,18.41 270 bottom
Q16  2N7002  [SOT-23]  2.79,22.86 270 bottom
R1  0R  [R0402]  7.62,30.1 270 bottom
R2  0R  [R0402]  7.62,30.86 270 bottom
R3  0R  [R0402]  7.62,31.62 270 bottom
R4  0R  [R0402]  7.62,32.51 270 bottom
R5  0R  [R0402]  24.38,1.78 0 bottom
R6  0R  [R0402]  7.11,42.8 270 bottom
R8  1k  [R0402]  8,36.83 180 bottom
R9  22R  [R0402]  40.64,24.77 270 bottom
R10  22R  [R0402]  40.64,26.04 270 bottom
R11  4.7K  [R0402]  3.11,13.72 270 bottom
R12  100K  [R0402]  3.11,14.73 270 bottom
R13  0R  [R0402]  3.81,44.83 90 bottom
R14  0R  [R0402]  3.81,42.29 90 bottom
R15  DNP  [R0402]  3.81,43.81 270 bottom
R16  22R  [R0402]  17.02,7.75 180 top
R17  22R  [R0402]  17.91,7.75 180 top
R18  DNP  [R0402]  3.81,43.05 270 bottom
R19  2K  [R0402]  15.37,16.76 0 top
R20  2K  [R0402]  13.34,12.19 270 top
R21  2K  [R0402]  13.34,13.08 270 top
R22  0R  [R0402]  30.23,50.8 180 bottom
R23  15K  [R0402]  14.86,12.7 180 bottom
R24  0R  [R0402]  23.62,3.56 0 bottom
R25  22R  [R0402]  11.81,13.97 0 bottom
R26  22R  [R0402]  13.34,13.97 0 bottom
R27  22R  [R0402]  14.86,13.97 0 bottom
R28  1M  [R0402]  6.22,36.83 0 bottom
R29  0R  [R0402]  34.8,1.52 0 top
R30  0R  [R0402]  6.99,5.71 180 top
R31  4.7K  [R0402]  33.15,4.45 270 top
R32  0R  [R0402]  16.13,18.92 180 top
R33  DNP  [R0402]  15.37,18.92 180 top
R34  0R  [R0402]  17.02,16.51 90 top
R35  4.7K  [R0402]  27.69,40.39 90 top
R36  4.7K  [R0402]  27.69,41.27 90 top
R37  470R  [R0402]  6.1,19.81 0 bottom
R38  10K  [R0402]  8.13,22.99 180 bottom
R39  0R  [R0402]  6.22,32.51 90 bottom
R40  0R  [R0402]  6.22,31.62 90 bottom
R41  0R  [R0402]  6.22,30.86 90 bottom
R42  0R  [R0402]  6.22,30.1 90 bottom
R43  470R  [R0402]  20.32,27.3 0 top
R44  470R  [R0402]  19.56,27.3 0 top
R45  100K_1%  [R0402]  29.97,46.23 270 top
R46  10M  [R0402]  19.05,11.94 270 top
R47  10M  [R0402]  20.51,11.18 270 top
R48  0R  [R0402]  32.77,19.56 0 top
R49  22K_1%  [R0402]  31.75,45.34 270 top
R50  4.7K  [R0402]  26.42,17.78 0 top
R51  4.7K  [R0402]  27.18,17.78 0 top
R52  0R  [R0402]  28.7,25.91 90 top
R53  0R  [R0402]  27.94,17.78 0 top
R54  0R  [R0402]  32.77,22.92 0 top
R55  0R  [R0402]  32.77,21.59 180 top
R56  DNP  [R0402]  13.34,34.54 270 top
R57  0R  [R0402]  23.62,10.92 180 bottom
R58  0R  [R0402]  24.38,5.46 180 bottom
R60  0R  [R0402]  42.67,19.56 270 bottom
R61  0R  [R0402]  40.51,19.56 270 bottom
R62  DNP  [R0402]  24.38,3.56 180 bottom
R63  DNP  [R0402]  23.62,5.46 0 bottom
R64  DNP  [R0402]  42.67,18.54 90 bottom
R65  DNP  [R0402]  40.51,18.54 90 bottom
R70  1.5K  [R0402]  36.39,21.21 270 top
R71  1K  [R0402]  36.39,20.45 90 top
R72  1.5K  [R0402]  34.99,21.21 270 top
R73  1K  [R0402]  34.99,20.45 90 top
R74  10M  [R0402]  21.21,7.49 90 top
R75  0R  [R0402]  30.35,14.35 0 top
R76  DNP  [R0402]  23.62,1.78 180 bottom
R77  DNP  [R0402]  13.34,33.78 270 top
R78  1k  [R0402]  21.21,6.6 90 top
R79  DNP  [R0402]  45.97,47.62 90 bottom
R80  DNP  [R0402]  24.38,10.92 180 bottom
R81  4.7K  [R0402]  45.97,48.64 270 bottom
R82  0R  [R0402]  31.11,14.35 0 top
R83  0R  [R0603]  28.19,15.49 90 top
R84  0R  [R0603]  28.19,14.1 90 top
R85  DNP  [R0402]  7.11,19.81 0 bottom
R86  DNP  [R0402]  8.13,19.81 0 bottom
R87  DNP  [R0402]  8.13,21.21 0 bottom
R89  DNP  [R0402]  16.89,18.92 0 top
R90  0R  [R0402]  29.97,45.34 270 top
R91  470R  [R0402]  34.54,4.45 270 top
R92  DNP  [R0402]  34.54,7.75 270 top
R93  470R  [R0402]  34.54,9.78 270 top
R94  DNP  [R0402]  34.92,13.08 270 top
R95  0R  [R0402]  21.84,27.3 180 top
R96  10K  [R0402]  45.97,46.86 270 bottom
R97  200K1%  [R0402]  45.59,43.94 180 bottom
R98  30K1%  [R0402]  46.35,43.94 0 bottom
R99  100K  [R0402]  45.97,46.1 270 bottom
R100  10K  [R0402]  12.83,28.32 180 top
R101  10K  [R0402]  21.08,27.3 0 top
R102  1k  [R0402]  3.17,36.58 270 bottom
R103  470k  [R0402]  3.17,32.51 90 bottom
R104  1M  [R0402]  3.17,37.34 90 bottom
R105  1k  [R0402]  3.17,25.27 270 bottom
R106  470k  [R0402]  3.17,20.45 90 bottom
R107  1M  [R0402]  3.17,26.8 90 bottom
R108  0R  [R0603']  35.05,16.51 180 top
R109  0R  [R0402]  8,50.8 180 bottom
R110  0R  [R0402]  24.51,50.8 180 bottom
R111  0R  [R0402]  26.42,52.58 0 bottom
R112  DNP  [R0402]  13.34,35.31 90 top
R113  0R  [R0402]  7.11,42.04 90 bottom
R114  0R  [R0402]  7.11,40.51 90 bottom
R117  0R  [R0402]  7.11,38.86 270 bottom
R118  0R  [R0402]  6.22,28.83 90 bottom
R119  0R  [R0402]  7.62,27.69 270 bottom
R120  0R  [R0402]  7.62,26.67 270 bottom
R121  0R  [R0402]  7.49,17.65 90 bottom
R122  0R  [R0402]  7.49,16.13 90 bottom
R123  0R  [R0402]  7.49,14.61 90 bottom
R124  0R  [R0402]  44.32,15.62 90 bottom
R125  4.7K  [R0402]  17.65,18.92 0 top
R126  DNP  [R0402]  18.41,18.92 0 top
R127  0R  [R0402]  44.32,16.51 90 bottom
R128  0R  [R0402]  44.32,17.4 90 bottom
R129  0R  [R0402]  33.4,30.99 270 top
R130  0R  [R0402]  33.4,32 270 top
R131  0R  [R0402]  33.4,33.15 270 top
R132  0R  [R0402]  35.05,38.73 270 top
R133  0R  [R0402]  35.05,40.26 270 top
R134  0R  [R0402]  35.05,41.78 270 top
R135  1k  [R0402]  2.41,5.59 180 bottom
R136  470k  [R0402]  4.45,13.97 180 bottom
R137  1M  [R0402]  3.94,5.59 0 bottom
R139  470k  [R0402]  4.57,38.1 270 bottom
R141  DNP  [R0402]  28.19,14.1 180 bottom
R142  1k  [R0402]  29.72,38.99 270 top
R143  470k  [R0402]  30.48,34.29 270 top
R144  1M  [R0402]  31.24,39.88 270 top
R145  0R  [R0402]  33.27,17.78 0 top
TP1  [TP-D45MIL]  14.61,6.99 0 bottom
TP2  [TP-D45MIL]  20.32,6.99 0 bottom
TP3  [TP-D45MIL]  16.51,6.99 0 bottom
TP4  [TP-D45MIL]  18.41,6.99 0 bottom
TP5  [TP-D45MIL]  42.93,35.69 0 bottom
TP8  [TP-D45MIL]  33.66,26.04 180 top
TP12  [TP-D45MIL]  40.64,20.95 0 bottom
TP13  [TP-D45MIL]  42.55,22.86 180 bottom
TP14  [TP-D45MIL]  42.55,24.77 180 bottom
TP15  [TP-D45MIL]  42.55,26.67 180 bottom
TP16  [TP-D45MIL]  42.55,20.95 180 bottom
TP17  [TP-D45MIL]  20.95,14.61 180 bottom
TP18  [TP-D45MIL]  19.05,14.61 180 bottom
TP19  [TP-D45MIL]  22.86,14.61 180 bottom
TP20  [TP-D45MIL]  18.41,8.89 0 bottom
TP21  [TP-D45MIL]  20.32,8.89 0 bottom
U1  EC21-A  [MODULE144P-1.3-32X29X2.4MM]  24.13,32.13 90 bottom
U3  STM32F412RG  [LQFP64]  20.95,35.56 180 top
U4  ALC5616  [QFN32G-0.4-4X4MM]  29.21,21.59 180 top
U5  ETA6003  [QFN16G-0.5-3X3MM@1]  16.26,13.72 180 top
U6  ETA3410  [DFN8G-0.5-2X2MM]  32.38,43.43 180 top
U8  MP28164  [QFN11-0.5-2X3MM]  43.43,45.85 0 bottom
U9  TXS0108E  [TSSOP20-0.65-6.5X4.4MM]  15.88,23.5 0 top
U11  XC6206P182MR  [SOT-23]  34.04,28.7 0 top
U$97  [OSHW_FILLX100_NOTEXT]  17.78,50.8 0 top
U$98  [SEEED-SILK--TNAME-160*153MIL]  23.5,52.07 0 top
X1  32.768KHZ  [X2-SMD-L2.0X1.2X0.55MM]  25.21,45.34 180 top
X3  8M  [RESONATOR3-SMD-3.6X1.3X0.8MM]  22.23,43.81 180 top

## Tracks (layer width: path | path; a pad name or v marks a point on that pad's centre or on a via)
5V  (via drill 0.2 pad 0.41, 0.25 pad 0.51, 0.3 pad 0.64)
  Top 0.254: U5.2 C3.1 | v13.72,18.03 13.97,17.78 15.11,17.78 15.37,18.03 R33.1
  Top 0.305: R95.1 v21.84,26.54
  Top 0.406: v13.72,18.03 13.46,18.03 12.19,19.3 12.19,23.62 v12.57,24
  Top 0.508: F1.2 14.61,9.65 14.99,9.27 16,9.27 16.26,9.53 15.24,9.53 15.11,9.65
  Top 0.61: 16.6,9.9 14.22,9.9 F1.2 | D1.1 16.55,9.9 C8.2 16.6,9.9 | 16.6,9.9 C7.2 v18.16,9.91 | C3.1 19.34,12.73 v19.3,12.76
  VDD_3V3 0.406: v12.57,24 12.32,24 11.94,24.38 11.94,25.78 12.7,26.54 v21.84,26.54
  other vias: 15.24,9.27 15.88,9.27 13.53,15.62 12.76,15.37
  pour VDD_3V3 (isolate 0.254, no thermals): 18.92,13.08 19.68,13.08 19.94,12.83 19.94,12.06 18.41,10.54 18.41,9.4 17.91,8.89 14.61,8.89 13.21,10.29 13.21,14.61 12.83,14.99 12.45,15.37 12.45,16.13 13.21,16.89 13.21,18.29 13.34,18.41 13.97,18.41 14.22,18.16 14.22,12.19 14.73,11.68 17.91,11.68 18.8,12.57 18.8,12.95
  pour Top (isolate 0.254, no thermals): 13.72,14.73 12.95,14.73 12.45,15.24 12.45,15.62 12.7,15.88 13.72,15.88 14.1,15.49 14.1,14.86 13.97,14.73
A4  (via drill 0.2 pad 0.41)
  Top 0.127: U3.20 16.8,37.81 v17.14,37.47 | v43.94,17.91 38.48,17.91 v38.1,17.53
  VDD_3V3 0.127: v38.1,17.53 35.69,17.53 34.92,18.29 34.92,24.89 29.27,30.54 29.27,35.31 26.86,37.72 17.4,37.72 v17.14,37.47
  Bottom 0.127: R128.2 v43.94,17.91
A5  (via drill 0.2 pad 0.41)
  Top 0.127: U3.21 16.54,37.31 v16.89,36.96
  VDD_3V3 0.127: v16.89,36.96 17.4,36.96 17.91,37.47 26.68,37.47 28.96,35.19 28.96,30.48 34.67,24.77 34.67,17.65 36.7,15.62 v38.86,15.62
  Bottom 0.127: R127.2 43.18,15.75 38.99,15.75 v38.86,15.62
A6  (via drill 0.2 pad 0.41)
  Top 0.127: U3.22 8.36,36.81 6.35,34.8 6.35,26.42 5.84,25.91 5.84,15.24 v6.48,14.61
  Bottom 0.127: R123.2 v6.48,14.61
A7  (via drill 0.2 pad 0.41)
  Top 0.127: U3.23 14.24,36.31 13.97,36.58 8.51,36.58 6.6,34.67 6.6,26.16 6.1,25.65 6.1,16.38 6.35,16.13 v6.48,16.13
  Bottom 0.127: R122.2 v6.48,16.13
AGND  (via drill 0.2 pad 0.41)
  Top 0.203: C37.1 33.84,19.94 34.04,19.75
  Top 0.254: U4.7 31.8,22.59 v31.81,22.61 | U4.18 26.3,22.59 25.91,22.99 24.77,22.99 24.64,22.86 C33.2 24.38,22.48 v24.26,22.35
  Top 0.305: C90.1 C94.1 32.57,13.9 D15.2 31.88,13.46 | C83.1 C85.1 C84.1 31.24,16.26 30.86,15.88 30.86,15.37 30.35,14.86 R75.1 29.97,14.73 29.72,14.99 | C51.1 C50.1 C49.1 | C54.1 33.53,22.04 v33.85,22.35 | C45.1 25.15,25.91 24,24.77 24,23.62 23.11,22.73 | 29.72,14.99 29.72,16.26 29.53,16.45 | 29.72,14.99 29.72,13.59
  Top 0.406: v31.24,23.75 31.24,24.64 C42.1 C53.1 C52.1
  VDD_3V3 0.305: v29.65,15.56 v26.29,15.56
  VDD_3V3 0.406: v31.24,23.75 31.8,23.19 31.8,22.62 v31.81,22.61 | v24.26,22.35 23.37,22.35 v23.11,22.61
  pour Top (isolate 0.127, rank 2, no thermals): 22.86,13.34 22.86,23.36 26.42,26.92 26.42,28.01 26.9,28.49 28.8,28.49 31.11,26.18 32.4,24.87 36.49,24.89 37.47,23.92 37.47,16.51 34.42,16.51 34.42,13.34
ANT_DIV
  Bottom 0.305: R109.1 C95.2 8,44.71 arc90 9.34,43.38 U1.35
ANT_GNSS
  Bottom 0.305: U1.47 24.53,49.51 C99.2 R110.1
ANT_MAIN
  Bottom 0.305: U1.49 C9.2 R22.1
ANT_POWR  (via drill 0.2 pad 0.41)
  Top 0.127: U3.33 17.2,29.02 v17.14,28.96 | v8.51,25.27 8.7,25.46 12.26,25.46 12.45,25.27 v13.08,25.27
  Bottom 0.127: v17.14,28.96 16.38,28.19 16.38,26.29 15.88,25.78 13.59,25.78 v13.08,25.27 | R105.2 v8.51,25.27
AP_READY
  Top 0.127: U3.9 20.7,34.74 16.51,30.54 16.51,28.19 17.48,27.22 U9.13
AP_READY_MODULE  (via drill 0.2 pad 0.41)
  Top 0.127: U9.8 17.5,21.69 v18.03,22.23
  Bottom 0.127: 35.43,17.15 U1.2 35.31,16.86 35.31,17.4 34.8,17.91 32.51,17.91 32.07,18.35 20.64,18.35 20.19,18.8 20.19,19.81 19.81,20.19 18.67,20.19 18.29,20.57 18.29,21.97 v18.03,22.23
AVDD
  Top 0.127: U4.6 31.97,22.19 32.26,22.48 32.26,22.8 R54.1 C53.2 C52.2
BAT_C  (via drill 0.2 pad 0.41)
  Top 0.254: U3.26 16.14,34.81 v16.64,35.31
  Top 0.381: v19.94,10.54 20.13,10.73 R47.2 C78.1 R46.1
  Bottom 0.254: v19.94,10.54 12.95,10.54 10.16,13.33 10.16,17.4 11.56,18.8 11.56,22.23 12.06,22.73 12.06,27.81 11.87,28 11.87,33.82 13.36,35.31 v16.64,35.31
BOOT0  (via drill 0.2 pad 0.41)
  Top 0.127: U3.60 25.88,37.31 24.51,35.94 v24.51,34.67 | v6.35,35.56 6.1,35.31 6.1,30.48 4.83,29.21 4.83,15.49 v4.95,15.37
  VDD_3V3 0.127: v24.51,34.67 7.24,34.67 v6.35,35.56
  Bottom 0.127: v4.95,15.37 2.92,15.37 2.73,15.18 R12.1 2.23,14.24 K1.4
BOOT1
  Top 0.127: R112.2 R56.1 14.45,33.81 U3.28
CD/DATA3
  Bottom 0.127: R24.1 R62.2 C61.1 25.97,3.94 D23.1 26.04,4.19 26.23,4.38 26.99,4.38 28.19,3.17 35.56,3.17 36.2,2.54 36.2,1.91 35.81,1.52 J2.T2
CODEC_PCM_CLK
  Bottom 0.127: R4.1 R39.1
CODEC_PCM_IN
  Bottom 0.127: R1.1 R42.1
CODEC_PCM_OUT
  Bottom 0.127: R2.1 R41.1
CODEC_PCM_SYNC
  Bottom 0.127: R3.1 R40.1
CPVDD
  Top 0.203: U4.15 28.21,24.18 27.88,24.51 27.88,25.84 27.94,25.91 | C35.2 C43.2 C45.2 27.94,25.91 | 27.94,25.91 R52.1
D19  (via drill 0.2 pad 0.41)
  Top 0.127: U3.55 25.39,34.81 25.02,35.18 v25.02,35.69
  Bottom 0.127: v25.02,35.69 24.64,35.31 21.72,35.31 21.34,34.92 17.65,34.92 16.89,35.69 13.27,35.69 11.56,33.98 v11.56,27.69 11.56,27.43 11.3,27.18 9.14,27.18 8.64,27.69 R119.2
D20  (via drill 0.2 pad 0.41)
  Top 0.127: U3.56 v25.91,35.31
  VDD_3V3 0.127: v8.38,26.54 14.22,32.38 21.46,32.38 v21.59,32.26
  Bottom 0.127: v25.91,35.31 25.78,35.31 22.73,32.26 v21.59,32.26 | R120.2 8.26,26.67 v8.38,26.54
D38  (via drill 0.2 pad 0.41)
  Top 0.127: v21.72,39.62 21.72,34.04 19.2,31.52 U3.37
  VDD_3V3 0.127: v21.72,39.62 v12.19,39.62
  Bottom 0.127: R117.2 11.43,38.86 v12.19,39.62
D39  (via drill 0.2 pad 0.41)
  Top 0.127: v22.23,40.01 22.23,34.04 19.7,31.52 U3.38
  VDD_3V3 0.127: v22.23,40.01 12.83,40.01 11.94,40.89 6.35,40.89 v6.22,41.02
  Bottom 0.127: R114.2 v6.22,41.02
DACREF
  Top 0.127: C54.2 R55.1 32.18,21.79 U4.5
DBG_RXD
  Bottom 0.203: U1.11 20.63,14.93 TP17.T
DBG_TXD
  Bottom 0.203: U1.12 19.33,14.88 TP18.T
DTR  (via drill 0.2 pad 0.41)
  Top 0.127: U9.3 14.25,22.2 v14.22,22.23
  Bottom 0.127: v14.22,22.23 14.61,22.61 16.38,22.61 16.89,23.11 16.89,27.69 17.91,28.7 35.05,28.7 36.73,30.38 U1.66
DTR_MODULE  (via drill 0.2 pad 0.41)
  Top 0.127: U9.18 14.25,27.2 14.99,27.94 14.99,28.83 14.1,29.72 12.95,29.72 12.19,30.48 12.19,31.5 11.81,31.88 11.81,34.92 v12.06,35.18 | U3.15 17.7,40.08 18.8,38.99 v18.8,35.69
  VDD_3V3 0.127: v18.8,35.69 18.54,35.94 12.32,35.94 12.06,35.69 v12.06,35.18
GND  (via drill 0.2 pad 0.41)
  Top 0.203: v16.51,8.89 17.02,8.89 17.46,9.34 20.51,9.34 21.21,10.03 21.21,14.22 | U3.18 14.53,38.81 | 2.87,19.05 J13.SS2 | D5.2 18.86,8.07 19.24,8.45 21.02,8.45 22.16,9.59 22.16,23.3 23.5,24.64 v23.5,26.41 C125.1 C70.1 C71.1 | 21.08,17.65 21.08,23.62 22.48,25.02 22.48,27.69 | U9.11 18.79,27.29 v18.8,27.3 | 16.51,14.36 16.51,14.35 16.51,13.97 U5.PAD | 16.01,13.97 15.62,13.97 15.51,14.08 U5.8 15.51,15.52 | D1.2 16.2,10.8 16.55,10.8 C8.1 16.73,10.67 C7.1 | C24.2 18.29,16.13 v17.65,15.49 | C47.1 C48.2 C46.2 v30.23,15.49 | C44.2 C41.2 C40.2 v24.26,18.92 | U4.PAD v28.57,22.23 | R108.1 35.05,13.34 R94.1 | D27.2 34.73,1.07 R29.2 | v40.51,1.91 40.51,1.52 40.19,1.2 C16.1 | U5.13 15.51,12.84 v15.88,13.21 | 21.08,17.65 20.7,18.03 | 21.21,14.22 21.21,17.53 21.08,17.65 | 21.21,14.22 21.08,14.1 | 21.08,14.1 20.7,13.72 | 21.08,14.1 20.83,14.1 20.57,13.84
  Top 0.254: C11.2 24.39,44.2 v24.19,44.01 | U6.6 32.25,43.68 v32.38,43.81 32.52,43.68 U6.3 | 37.87,38.48 J14.4 | U6.1 32.63,42.68 v32.38,42.93 | U3.12 19.2,42.38 v19.3,42.48 | U3.18 15.86,38.81 v16.38,38.29 | C31.1 C30.1 v14.1,37.53 | C68.1 C32.1 C1.1 | v8.64,30.61 10.23,30.61 J12.4 | v19.94,9.84 19.43,10.35 C25.2 | 16.01,13.97 U5.PAD | U5.13 15.51,11.82 | 15.51,11.82 15.51,11.43 15.51,11.19 | 15.51,11.19 15.51,10.91 15.62,10.79 15.62,10.92 16.51,10.92 | 15.51,11.82 15.24,11.56 | 15.51,11.19 15.24,10.92 | 15.24,11.18 15.24,11.3 15.37,11.43 15.37,11.3 | 17.65,10.67 17.5,10.82 C8.1 16.54,10.82 16.38,10.67 15.11,10.67 | U5.10 15.62,13.97 | R32.2 v16.13,19.62 | R126.1 18.8,19.31 19.3,19.81 20.19,19.81
  Top 0.279: U5.6 16.51,14.36 v16.64,14.22 | U5.10 13.97,13.97
  Top 0.305: v34.92,10.92 34.16,10.92 Q10.2 | C65.1 14.35,19.31 v14.1,19.56 | C68.1 12.95,30.36 v13.08,30.23 | C1.1 12.7,32.26 | U6.6 30.74,43.68 30.26,44.16 C105.1 | R92.1 35.43,7.75 36.26,6.92 v36.26,6.41 | C3.2 20.95,13.46 | C71.1 C70.1 C125.1 24,26.8 23.62,26.42 | C70.1 24.77,26.42 | R20.2 v12.45,12.19 | R21.2 12.57,13.08 v12.45,12.95 | 15.24,11.18 15.24,10.92 | 15.24,10.92 15.37,10.79 | 15.24,10.92 15.24,10.86 15.11,10.73 | 16.2,10.8 16.14,10.8 15.51,11.43 | U3.63 27.76,38.81 v27.94,38.99 | v4.13,34.42 4.19,34.35 4.19,33.78 3.5,33.09 J12.SS2 2.49,32.77 2.29,32.77 1.97,32.45 v1.97,31.75 | 16.16,19.27 R32.2 | J16.SS1 44.52,19.12 v43.81,18.41 | C139.2 17.56,42.96 v18.03,42.48 | v19.3,42.48 v19.31,42.48 C118.1 C119.1 | C23.2 20.77,45.59 v20.95,45.78 | C38.1 v26.99,44.51 26.67,44.2 C39.1 C10.2 | X3.2 v22.23,45.02 | J11.4 12.02,44.66 v12.06,44.7 12.83,45.47 LED2.2 | C133.2 v34.16,39.5 | 31.62,39.75 R144.1 31.62,40.26 31.37,40.51 | 31.62,39.75 v31.62,39.5 | v31.62,39.5 v31.62,39.49 C143.2 32.13,39.5 | C135.2 v34.16,41.02 | R112.1 12.83,35.31 v12.57,35.56 | C31.1 v12.32,37.53 | R94.1 35.69,13.08 v35.81,12.95 | v31.62,39.5 32.13,39.5 | 32.13,39.5 32.38,39.5 | 31.62,39.75 32.25,39.75 32.26,39.75 | C134.2 34.67,37.28 v34.8,37.15 | J14.4 36.56,38.66 v36.45,38.54
  Top 0.381: J13.SS2 3.19,19.12 3.62,19.12 | C78.2 R47.1 21.08,11.18 | C78.2 20.89,12.25 v20.64,12.51 20.38,12.76 v20.38,12.89 20.54,13.05 C3.2 | C78.2 21.08,11.94
  Top 0.406: C142.2 29.21,29.59 v28.83,29.97 | 3.19,19.12 3.19,18.21 v3.24,18.16 | R144.1 v31.62,40.89 | C129.2 v36.2,33.15 | C127.2 v36.26,32 | C128.2 35.56,30.99 v35.69,31.11
  Top 0.508: 13.97,13.97 13.43,13.97 C4.2
  Bottom 0.127: D10.2 24.45,7.62 v22.48,9.59 | D11.2 v27.56,6.1 26.42,6.1 | D8.2 v27.56,6.86
  Bottom 0.203: C79.2 2.57,27.91 | 2.57,27.91 v3.17,27.3 3.56,26.92 R107.1 C93.2 | 2.57,27.91 2.57,27.4 v2.54,27.37 | 23.24,27.56 23.37,27.56 23.79,27.13 | U1.105 24.13,27.05 C125.1 23.79,27.13 | U1.106 23.79,27.13 | C59.2 v17.65,14.99 v17.65,15.49 | v28.57,22.23 28.57,23.58 U1.109 29,24 29.72,24 29.84,23.88 v29.84,22.23 | J2.PAD1 31.37,14.35 v30.23,15.49 | C60.2 40.9,16.58 D19.2
  Bottom 0.254: 40.83,42.61 C106.1 | 39.64,42.98 39.37,42.98 39.37,43.56 v39.37,43.62 | U1.93 19.33,37.11 19.05,36.83 | v16.38,38.29 16.38,36.83 14.83,36.83 U1.94 14.49,37.13 v14.1,37.53 | 13.34,33.66 14.45,33.66 U1.98 | U1.102 14.53,29.92 v14.61,29.84 | Q14.2 4.45,33.66 | 39.33,22.18 v39.37,22.23 | C12.2 26.03,1.4 26.04,1.4 D7.2 26.04,1.14 26.16,1.02 v26.42,1.02 | C17.2 v25.65,5.84 25.72,5.91 D22.2 | 26.42,6.1 26.16,6.1 | 26.16,6.1 26.04,5.97 D22.2 | D22.2 26.09,5.91 26.16,5.84 | 26.16,5.84 26.8,5.21 27.3,5.21 27.43,5.33 D12.2 | 26.16,5.84 26.16,6.1 | C6.2 v25.65,11.3 25.72,11.37 D21.2 | U8.9 v43.18,45.85 | U8.5 v43.7,45.1 v43.69,45.09 | C55.2 44.04,43.59 43.81,43.81 v43.81,44.07 | R98.2 v46.35,43.05 | C56.1 v46.74,45.09 | C61.2 25.97,3.17 D23.2 25.59,3.11 25.53,3.05 v25.53,2.79 C61.2
  Bottom 0.305: TP19.T 22.86,14.48 v22.35,13.97 | 8.91,22.18 v8.89,22.16 8.32,22.16 8.26,22.23 | R87.1 8.13,22.1 8.26,22.23 | 8.26,22.23 v8.26,22.16 | R38.1 8.13,22.35 8.26,22.23 | Q1.2 8.26,22.23 | U1.112 14.53,23.95 v13.97,24.51 | U1.107 14.53,27.25 13.72,28.07 v13.72,29.34 | 14.05,33.73 U1.98 15.95,33.73 16.13,33.91 17.02,33.91 17.27,33.66 v17.27,33.4 17.6,33.73 U1.97 | C13.1 44.04,48.23 43.43,47.62 43.43,46.1 v43.18,45.85 | v43.69,45.09 43.69,44.96 43.56,44.83 43.56,44.32 v43.81,44.07 | C15.2 40.04,43.4 | 40.04,43.4 v40.39,43.05 C106.1 | 40.01,43.66 C15.2 | C15.2 40.01,43.69 | 40.01,43.69 39.5,43.69 39.37,43.56 | 39.37,43.69 39.37,43.56 | 44.04,43.59 44.74,43.59 v44.83,43.69 | v47.37,38.73 46.48,38.73 46.04,38.29 C77.- 46.04,37.91 46.48,37.47 v47.37,37.47 | v47.37,40.64 46.61,40.64 46.1,41.15 C113.- 46.04,41.34 46.86,42.16 | C14.1 40.07,36.95 D28.2 | C19.2 14.1,14.48 14.61,14.99 v14.61,14.92 | C20.2 12.57,14.54 v12.38,14.73 | C60.2 40.9,17.27 v40.77,17.14 | C115.2 v5.84,27.24 C64.2 | C92.2 3.78,16.29 v3.37,16.7 | C57.2 6.22,39.24 v5.78,39.24 | C63.2 6.48,41.53 v6.03,41.53 | R104.1 v3.56,37.72 C91.2 | 4.45,33.66 4.45,34.1 v4.13,34.42 | Q5.2 v8.64,33.66 | C114.2 v8,29.34 | U1.22 9.34,26.48 v8.76,25.91 | R12.2 3.75,14.73 v3.94,14.92 | D20.2 43.05,16.57 C18.2 43.05,17.72 43.75,18.41 v43.81,18.41 | U1.103 33.96,27.13 v34.04,27.05 | U1.99 33.48,30.53 v32.13,31.88 | U1.95 33.98,33.73 v34.29,34.04 | U1.93 U1.92 | U1.89 15.63,40.33 v16.26,40.96 | U1.46 23.23,46.05 v23.5,45.78 | U1.36 12.04,44.68 v12.06,44.7 | v7.49,44.07 v7.5,44.07 C22.1 7.62,43.56 7.87,43.31 | U1.88 19.33,42.46 v19.3,42.48 | v34.16,39.5 33.73,39.93 U1.85 33.2,40.33 v32.64,40.89
  Bottom 0.305: U1.56 39.19,43.38 39.37,43.56 | 40.83,42.61 40.44,42.61 40.39,42.67 | 40.01,43.69 39.5,44.2 | 40.04,43.4 39.84,43.4 39.5,43.05 | 46.86,42.16 v47.37,42.16 | 46.86,42.16 46.48,42.16 46.35,42.04 | 7.87,43.31 8.13,43.05 v8.38,43.05 | 7.87,43.31 7.87,43.56 7.62,43.81 7.62,44.07 7.49,44.2
  Bottom 0.406: U1.19 9.25,22.58 8.89,22.23 8.89,22.2 8.91,22.18 | U1.72 39.01,22.58 v39.37,22.23
  other vias: 15.56,7.24 40.39,36.58 40.89,36.58 9.53,49.53 11.43,49.53 13.34,49.53 15.88,49.53 17.14,49.53 20.45,49.53 23.5,50.16 6.35,49.53 5.84,51.56 6.35,53.34 8.26,53.34 13.34,53.34 13.34,51.44 9.53,50.8 9.53,53.34 15.24,52.07 19.18,50.8 22.86,53.34 22.61,50.16 24.13,53.98 27.3,53.98 27.3,52.07 27.3,50.16 23.5,51.44 29.21,50.8 28.57,52.07 28.07,49.4 31.11,49.53 31.11,50.8 29.21,53.34 31.11,53.34 36.2,53.34 36.2,50.8 36.2,49.53 33.66,49.53 39.37,50.16 28,45.15 40.39,42.61 40.89,39.69 41.4,39.69 32.77,45.09 33.66,45.09 24.89,38.99 24.13,40.01 24.77,36.83 14.61,30.73 4.06,21.21 5.08,8.89 6.48,6.1 16.13,6.1 22.61,11.81 22.48,27.94 15.24,24.51 10.79,15.62 34.92,11.68 38.61,6.41 37.21,6.41 34.48,6.16 41.91,1.14 42.67,6.99 45.72,6.99 40.39,7.62 45.09,20.7 45.09,11.43 45.09,24.13 45.09,26.8 45.09,29.21 42.67,4.95 23.11,31.11 24.13,30.86 26.67,31.11 26.67,29.97 28.57,27.3 33.78,23.24 28.83,2.41 28.83,1.02 20.45,10.03 5.08,50.16 7.37,52.83 6.99,50.8 5.71,52.7 14.61,50.8 16.51,50.8 15.88,53.34 18.41,53.34 36.2,51.82 37.59,49.53 39.37,53.34 40.64,51.44 15.88,14.22 16.26,13.72 6.99,4.45 8.26,3.81 20.57,22.23 22.35,22.23 22.35,26.04 22.99,24 18.41,23.75 20.32,23.75 26.42,49.4 39.37,52.07 44.58,48.64 44.58,48.13 12.64,32.26 29.97,41.27 29.97,40.39 37.72,47.37 47.37,35.18 47.37,32 12.64,18.03 12,18.03 24.26,19.43 28.19,20.57 30.1,20.57 32.13,46.23 18.16,15.49 18.16,14.99 41.91,11.43 6.48,15.43 6.48,16.83 6.48,13.91 3.05,6.73 6.29,37.97 5.97,44.45 45.72,14.35 46.99,15.62 18.03,30.86 32.64,39.62 33.72,37.15 4.45,5.97
  pour Top (isolate 0.203, rank 6): -0.64,-0.64 48.9,-0.64 48.9,55.12 -0.64,55.12
  pour Bottom (isolate 0.203, rank 6): -0.64,55.12 -0.64,-1.91 0.64,-1.91 0.64,-0.64 48.9,-0.64 48.9,55.12
  pour GND (isolate 0.203, rank 6): -0.64,-0.64 -0.64,-1.27 0.64,-1.27 0.64,-0.64 48.9,-0.64 48.9,55.12 -0.64,55.12
  pour Bottom (isolate 0.254, no thermals): 39.75,36.96 41.1,36.96 41.27,36.78 41.27,36.48 40.99,36.2 39.93,36.2 39.75,36.37
  pour Bottom (isolate 0.254, no thermals): 39.88,40.26 41.15,40.26 41.53,39.88 41.53,39.37 41.27,39.12 39.75,39.12 39.62,39.24 39.62,40.13 39.75,40.26
  pour Top (isolate 0.254, no thermals): 17.4,16.76 17.77,16.77 18.03,16.76 18.54,16.76 18.8,16.51 18.8,15.49 18.16,14.86 17.53,14.86 17.4,14.99 17.4,16.13 17.14,16.38 17.14,16.64 17.27,16.76
  pour Top (isolate 0.254, no thermals): 20.57,13.97 21.08,13.97 21.21,13.84 21.21,10.54 21.08,10.41 20.57,10.41 20.45,10.54 20.45,12.19 20.19,12.45 20.19,13.84 20.32,13.97
  pour VDD_3V3 (no thermals): 8.13,18.29 12.54,18.29 12.83,18 12.83,17.14 12.01,16.32 12.01,15.36 12.83,14.54 12.83,8.76 9.21,8.76 6.22,11.75 6.22,19.53 6.76,20.07 23.75,20.07 25.02,18.8 25.02,18.67 23.5,17.14 22.99,17.14 20.83,19.3 8.26,19.3 8,19.05 8,18.41
  pour Top (isolate 0.254, no thermals): 24.38,20.83 24.26,20.83 24,20.57 24,18.92 24.26,18.67 24.64,18.67 24.77,18.8 24.77,20.7 24.64,20.83
  pour Top (isolate 0.254, no thermals): 30.1,43.81 27.94,43.81 27.69,44.07 27.69,44.96 27.81,45.09 30.23,45.09 30.35,44.96 30.35,44.07
  pour Top (isolate 0.254, no thermals): 31.88,48.01 31.88,45.34 32.26,44.96 33.66,44.96 33.78,45.09 33.78,48.01 33.66,48.13 32,48.13
  pour VDD_3V3 (isolate 0.254, rank 2, no thermals): 19.43,15.37 19.43,14.55 16.82,11.94 14.88,11.94 14.48,12.34 14.48,14.99 14.73,15.24 15.01,15.24 15.43,15.66 19.14,15.66
  pour Top (isolate 0.254, no thermals): 21.08,18.03 21.08,19.51 20.9,19.68 20.45,19.68 20.32,19.56 20.32,18.41 20.83,17.91 20.95,17.91
GRO_POWR  (via drill 0.2 pad 0.41)
  Top 0.127: U3.29 16.55,33.31 v16.64,33.4 | v5.59,33.27 5.84,33.02 5.84,30.61 4.57,29.34 4.57,7.37 3.17,5.97 v1.78,5.97
  VDD_3V3 0.127: v5.59,33.27 6.1,32.77 12.83,32.77 13.46,33.4 v16.64,33.4
  Bottom 0.127: v1.78,5.97 R135.2
I2C1_SCL  (via drill 0.2 pad 0.41)
  Top 0.127: U3.61 25.82,37.81 25.53,38.1 25.53,40.89 25.91,41.27 v26.42,41.27 R36.1 | R134.2 v34.67,42.29
  Bottom 0.127: v26.42,41.27 27.18,42.04 34.42,42.04 v34.67,42.29
I2C1_SDA  (via drill 0.2 pad 0.41)
  Top 0.127: U3.62 25.95,38.31 25.78,38.48 25.78,40.13 26.04,40.39 v26.8,40.39 R35.1 | R133.2 34.16,40.26 33.53,39.62 v33.53,38.86
  Bottom 0.127: v26.8,40.39 26.8,41.27 27.18,41.66 30.35,41.66 30.73,41.27 30.73,39.37 31.11,38.99 33.4,38.99 v33.53,38.86
I2C_POWR  (via drill 0.2 pad 0.41)
  Top 0.127: U3.25 16.01,35.31 v17.27,36.58 | R142.2 28.83,38.99 v28.7,38.86
  Bottom 0.127: v28.7,38.86 28.32,38.48 18.03,38.48 17.53,37.97 17.53,36.83 v17.27,36.58
I2C_SCL  (via drill 0.2 pad 0.41)
  Top 0.127: U4.26 28.21,19.19 28.07,19.05 27.56,19.05 27.18,18.67 26.54,18.67 | 26.54,18.67 26.42,18.67 | 26.42,18.67 26.29,18.67 | 26.29,18.67 26.16,18.67 v26.04,18.8 | R50.1 26.42,18.54 | 26.42,18.54 26.42,18.67 | 26.29,18.67 26.42,18.54 | 26.42,18.54 26.54,18.67
  VDD_3V3 0.127: v26.04,18.8 24.38,20.45 6.73,20.45 4.32,22.86 4.32,33.15 2.54,34.92 2.54,45.27 2.79,45.53 2.83,45.56 3.31,46.04 v16.76,46.04
  Bottom 0.127: v16.76,46.04 16.76,47.5 U1.41
I2C_SDA  (via drill 0.2 pad 0.41)
  Top 0.127: U4.27 28.61,19.09 v28.26,18.73 27.75,18.73 R51.1
  VDD_3V3 0.127: v18.03,46.35 17.91,46.48 3.22,46.48 2.29,45.54 2.29,34.8 4.06,33.02 4.06,22.73 6.6,20.19 24.26,20.19 25.53,18.92 25.53,18.67 25.78,18.41 26.29,18.41 26.61,18.73 v28.26,18.73
  Bottom 0.127: U1.42 v18.03,46.36 v18.03,46.35
INT  (via drill 0.2 pad 0.41)
  Top 0.127: U9.20 12.95,27.82 R100.1 12.45,27.94 11.94,28.45 11.94,31.37 11.56,31.75 v11.56,35.43 | U3.14 18.2,39.96 19.3,38.86 v19.3,35.69
  VDD_3V3 0.127: v19.3,35.69 19.3,35.81 18.92,36.2 12.06,36.2 11.56,35.69 v11.56,35.43
JD1  (via drill 0.2 pad 0.41)
  Top 0.127: U4.1 31.68,20.19 v31.75,20.26 | v22.61,7.62 21.72,7.62 R74.2 20.83,6.73 R78.1
  VDD_3V3 0.127: v22.61,7.62 24.77,9.78 24.77,16.64 25.27,17.14 27.05,17.14 27.24,17.34 28.96,17.34 31.75,20.13 v31.75,20.26
JTCK-SWCLK  (via drill 0.2 pad 0.41)
  Top 0.127: U3.49 24.45,31.81 23.5,32.77 23.5,38.73 v23.75,38.99
  VDD_3V3 0.127: v23.75,38.99 23.75,39.12 22.48,40.39 12.95,40.39 12.06,41.27 8.26,41.27 v4.7,44.83
  Bottom 0.127: R13.1 v4.7,44.83
JTMS-SWDIO  (via drill 0.2 pad 0.41)
  Top 0.127: U3.46 23.7,31.67 23.11,32.26 v23.11,38.99
  VDD_3V3 0.127: v4.32,41.91 6.99,39.24 22.86,39.24 v23.11,38.99
  Bottom 0.127: R14.1 4.19,42.03 v4.32,41.91
LED_RGB  (via drill 0.2 pad 0.41)
  Top 0.203: 13.72,42.15 LED2.3
  Top 0.254: U3.27 17.16,34.31 17.78,34.92 17.78,38.61 v17.53,38.86 | v13.91,38.86 13.91,41.99 LED2.3
  Bottom 0.254: v17.53,38.86 v13.91,38.86
M_POWER  (via drill 0.2 pad 0.41)
  Top 0.127: U3.57 28.06,35.81 28.7,36.45 31.5,36.45 31.81,36.13 v31.81,35.31 | v41.53,35.81 42.04,36.32 42.04,42.16 41.66,42.55 41.66,45.09 43.43,46.86 43.43,48.26 44.2,49.02 v46.35,49.02 | v12.57,33.15 13.46,33.15 13.72,33.4 R77.1
  Bottom 0.127: v41.53,35.81 39.5,35.81 39.12,36.2 36.96,36.2 36.07,35.31 v31.81,35.31 26.67,35.31 26.16,34.8 25.65,34.8 22.61,31.75 15.11,31.75 14.61,32.26 13.46,32.26 v12.57,33.15 | R81.2 v46.36,49.02 v46.35,49.02
MIC+  (via drill 0.2 pad 0.41)
  Top 0.127: U4.3 31.71,20.99 v32,20.7 | 36.2,23.4 C81.2 36.39,23.18 36.01,22.8 v36.01,22.73
  Bottom 0.127: v32,20.7 32.58,20.13 33.84,20.13 34.29,20.58 34.29,21.81 34.83,22.35 35.62,22.35 v36.01,22.73
MIC-  (via drill 0.2 pad 0.41)
  Top 0.127: U4.4 31.95,21.39 v32.13,21.21 | C82.2 35.02,23.21 35.02,23.15 v35.43,22.73
  Bottom 0.127: v32.13,21.21 32.38,20.95 32.38,20.65 32.65,20.38 33.72,20.38 34.04,20.7 34.04,21.92 34.72,22.61 35.31,22.61 v35.43,22.73
MIC_N  (via drill 0.2 pad 0.41)
  Top 0.127: R72.2 34.73,21.21 34.73,21.75 C82.1 35.02,22.04 35.56,22.04 v35.62,21.97 | C84.2 C85.2 C83.2 v33.78,15.49
  Bottom 0.127: v33.78,15.49 33.91,15.62 37.21,15.62 37.45,15.86 37.45,18.05 36.07,19.43 36.07,21.53 v35.62,21.97
MIC_P  (via drill 0.2 pad 0.41)
  Top 0.127: R70.1 36.64,21.21 36.64,21.75 36.51,21.88 | 36.51,21.88 C81.1 36.77,22.39 v36.77,22.48 | 36.51,21.88 36.51,21.91 36.39,22.04 | v33.91,14.73 33.28,14.73 C90.2 C94.2 31.82,14.73 | 31.82,14.73 D15.1 | 31.82,14.73 R82.1
  Bottom 0.127: v36.77,22.48 36.32,22.04 36.32,19.56 37.71,18.17 37.71,15.74 37.34,15.37 34.54,15.37 v33.91,14.73
MICBIAS
  Top 0.127: R48.2 C37.2 34.06,18.64 36.65,18.64 36.89,18.89 36.89,20.38 36.7,20.45 R71.2
MICVDD
  Top 0.203: U4.31 30.21,18.94 C51.2 C50.2 C49.2 R145.1
N$1
  Bottom 0.127: R1.2 8.26,30.1 9.27,29.08 U1.24
N$2
  Bottom 0.127: U1.25 9.62,30.38 9.02,30.99 8.13,30.99 R2.2
N$3
  Bottom 0.127: U1.26 8.06,31.68 R3.2
N$4
  Bottom 0.127: U1.27 8.47,32.98 R4.2
N$5
  Bottom 0.127: R37.1 6.1,21.21 5.46,21.84 5.4,21.91 Q1.3
N$6  (via drill 0.2 pad 0.41)
  Top 0.127: J3.3 30.97,8.28
  Top 0.203: 30.2,8.28 J3.3 28.93,8.28 28.57,8.64 28.57,10.29 arc90 28.32,10.54 27.81,10.54 arc-90 27.56,10.79 27.56,10.92 arc-90 27.81,11.18 28.32,11.18 arc90 28.57,11.43 v28.57,12.06 | R84.2 28.8,14.13 v29.21,14.54
  Bottom 0.203: v28.57,12.06 29.34,12.06 29.59,12.32 29.59,14.35 29.4,14.54 v29.21,14.54
N$7
  Bottom 0.127: U1.70 39.84,25.18 R9.1
N$8
  Bottom 0.127: U1.69 39.81,26.48 R10.1
N$9
  Top 0.127: R43.2 20.32,26.57 D6.-
N$10  (via drill 0.2 pad 0.41)
  Top 0.127: v15.49,43.05 15.49,42.16 LED2.4
  VDD_3V3 0.127: v8,42.55 14.99,42.55 v15.49,43.05
  Bottom 0.127: C22.2 R6.2 7.75,42.55 v8,42.55
N$11
  Bottom 0.127: Q5.1 7.87,36.32 R8.1 C67.1 R28.2
N$13
  Bottom 0.305: R22.2 C34.2 ANT4.D
N$14
  Top 0.127: D14.+ 32.96,4.25 R31.2
N$15  (via drill 0.2 pad 0.41)
  Top 0.203: 24.17,8.68 J3.4 24.52,9.27 24.89,9.27 27.24,11.62 v28.13,11.62 | R83.2 28.8,15.46 v29.21,15.05
  Bottom 0.203: v28.13,11.62 29.52,11.62 30.01,12.11 30.01,14.44 29.46,14.99 29.27,14.99 v29.21,15.05
N$16
  Bottom 0.127: Q5.3 5.84,36.07 4.19,37.72 R139.1 4.19,38.73 3.56,39.37 Q4.1
N$17
  Top 0.152: U6.5 31.25,44.18 30.36,45.08 R90.1
N$18
  Top 0.203: U3.31 13.77,32.31 C1.2
N$19
  Top 0.203: U3.47 24.2,28.65 24,28.45 C125.2
N$20
  Bottom 0.127: J4.3 R15.1 R13.2
N$21
  Bottom 0.127: J4.4 2.57,41.81 3.05,42.29 R14.2 R18.1
N$22
  Top 0.127: D16.- 15.28,17.23 R19.1
N$23
  Top 0.127: 15,14.69 15.11,14.8 15.11,16.13 R19.2 | 15,14.69 U5.9 | 15,14.69 15,14.5 14.99,14.48
N$24  (via drill 0.2 pad 0.41)
  Bottom 0.406: TP1.T v14.61,5.97
  pour Top (isolate 0.203, no thermals): 15.37,3.81 16,3.81 16,5.33 15.37,5.97 15.11,5.97 14.86,6.22 14.86,7.49 13.08,7.49 13.08,5.97 13.97,5.08 14.99,5.08 15.37,4.7
N$25
  Top 0.127: U5.7 16.01,18.42 R32.1 R33.2
N$26
  Top 0.203: 18.78,14.47 18.8,14.48
  Top 0.279: U5.3 18.28,13.97 18.41,14.1 | U5.4 18.3,14.47 | 18.3,14.47 18.41,14.47 | 18.41,14.47 18.67,14.47 18.78,14.47 | 18.41,14.1 18.41,14.29 | 18.41,14.29 18.41,14.35 | 18.41,14.35 18.41,14.47 | 18.3,14.47 18.41,14.35 | 18.41,14.29 18.54,14.41 | 18.41,14.1 18.67,14.35
  Top 0.61: 18.67,14.47 19.05,14.85 L6.1
N$27
  Top 0.127: U5.11 14.1,13.47 R21.1
N$28  (via drill 0.3 pad 0.64)
  Top 0.203: 17.13,11.44 17.27,11.43 17.02,11.43 | 17.02,11.43 16.26,11.43 16.01,11.68 U5.14 | U5.16 17.01,11.44 17.02,11.43
  Top 0.305: 18.66,11.44 18.66,11.19 C25.1
  Top 0.406: 17.13,11.44 18.66,11.44 | R46.2 18.66,11.44 | 18.66,11.44 18.66,10.3 v19.05,9.91
  Top 0.61: J1.+ v41.66,3.56
  VDD_3V3 0.813: v19.05,9.91 19.05,7.67 22.03,4.7 40.51,4.7 v41.66,3.56
  Bottom 0.406: TP20.T 18.41,9.02 19.05,9.65 v19.05,9.91
N$29
  Top 0.127: R20.1 14.49,12.97 U5.12
N$31
  Bottom 0.127: R11.1 2.73,13.15 3.17,12.7 3.17,10.41 4.12,9.47 K1.2
N$33
  Bottom 0.127: J2.T1 34.76,2.19 34.04,2.92 28.07,2.92 27.81,3.17 26.92,3.17 26.04,2.29 D7.1 25.97,2.16 C12.1 R5.1 R76.2
N$34
  Bottom 0.127: J2.T8 34.76,12.41 33.4,11.05 30.48,11.05 29.9,10.47 D21.1 25.21,10.47 C6.1 R80.2 | R80.2 | R57.1 R80.2
N$37
  Bottom 0.305: U8.10 41.92,46.35 41.66,46.61
  Bottom 0.61: 41.66,46.61 41.47,46.8 41.4,46.86 41.26,47 L3.1
N$40
  Top 0.127: J14.3 36.47,40.66 36.2,40.39 36.2,39.49 R132.1 C134.1
N$41
  Bottom 0.305: U8.8 41.79,45.35 41.78,45.34
  Bottom 0.61: L3.2 41.65,45.2 41.78,45.34
N$43
  Top 0.127: J14.2 36.56,42.66 36.2,42.29 36.2,41.02 R133.1 C133.1
N$44
  Top 0.279: U5.5 17.01,15.95 16.67,16.29 16.64,16.32 R34.1
N$45
  Top 0.127: J14.1 36.53,44.66 36.32,44.45 36.32,42.8 35.44,41.91 R134.1 C135.1
N$46
  Bottom 0.305: U8.6 44.81,44.6 45.09,44.32 R97.2 R98.1
N$47  (via drill 0.2 pad 0.41)
  Top 0.127: v8.26,42.04 8.7,42.48 8.76,42.55 8.87,42.66 J11.3
  Bottom 0.127: v8.26,42.04 R113.1 C63.1
N$48
  pour Top (isolate 0.127, no thermals): 33.15,43.05 33.15,43.31 33.78,43.31 34.04,43.56 35.81,43.56 35.81,42.8 34.04,42.8 33.78,43.05
N$49  (via drill 0.2 pad 0.41)
  Top 0.305: R45.1 30.99,46.23 31.37,45.85 R49.2 v30.99,45.34 | U6.4 33.77,44.18 v33.91,44.32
